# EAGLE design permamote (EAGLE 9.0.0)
AUTHOR: NEAL JACKSON; REV: B; TITLE: PERMAMOTE

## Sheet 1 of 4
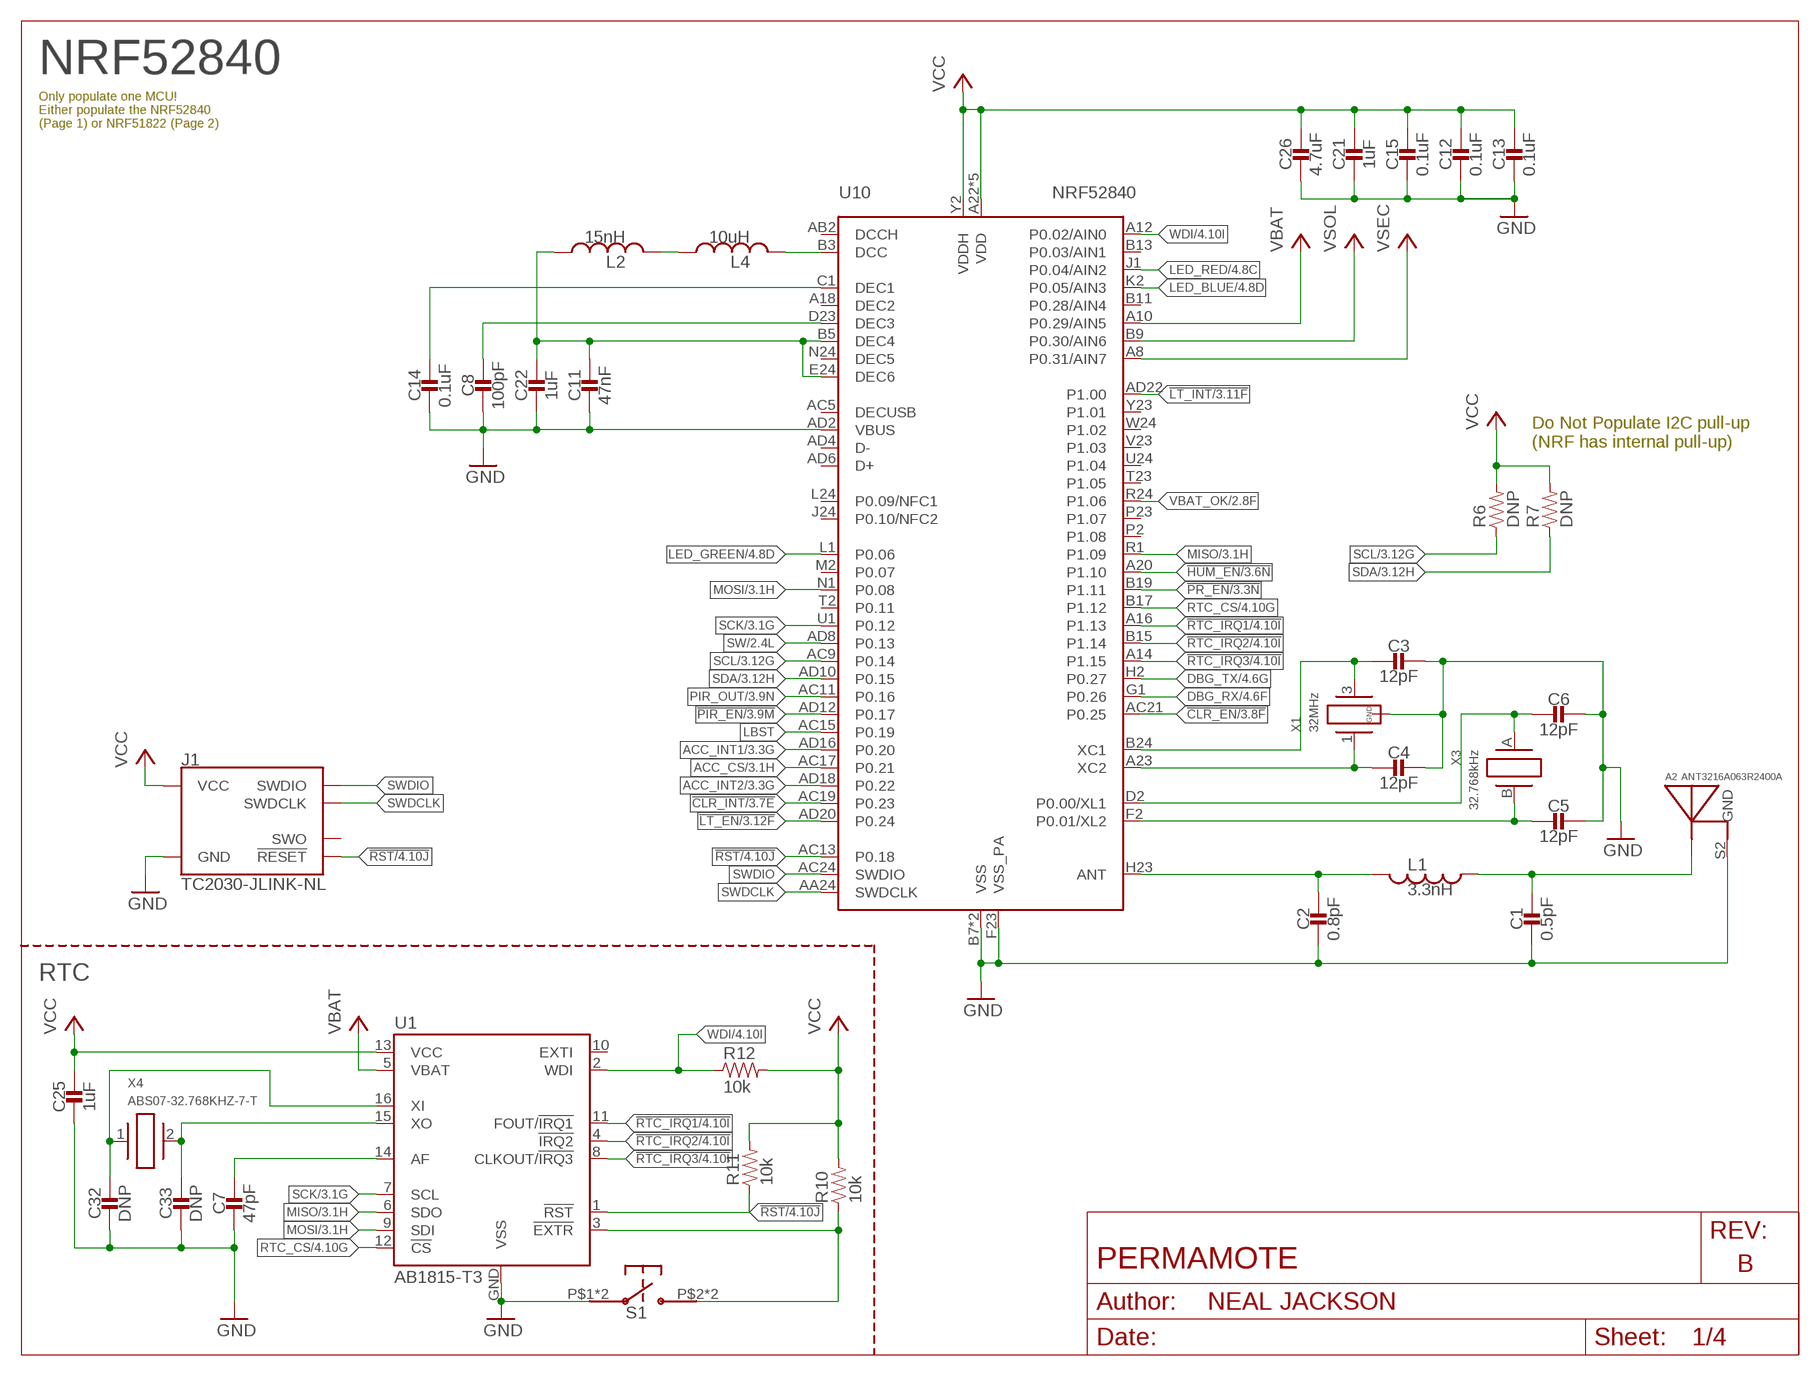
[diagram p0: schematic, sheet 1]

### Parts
A2  ANT3216A063R2400A  [ANT3216A063R2400A]
C1  0.5pF  CAPACITOR0402_CAP  [0402_CAP]
C2  0.8pF  CAPACITOR0402_CAP  [0402_CAP]
C3  12pF  CAPACITOR0402_CAP  [0402_CAP]
C4  12pF  CAPACITOR0402_CAP  [0402_CAP]
C5  12pF  CAPACITOR0402_CAP  [0402_CAP]
C6  12pF  CAPACITOR0402_CAP  [0402_CAP]
C7  47pF  CAPACITOR0402_CAP  [0402_CAP]
C8  100pF  CAPACITOR0402_CAP  [0402_CAP]
C11  47nF  CAPACITOR0402_CAP  [0402_CAP]
C12  0.1uF  CAPACITOR0402_CAP  [0402_CAP]
C13  0.1uF  CAPACITOR0402_CAP  [0402_CAP]
C14  0.1uF  CAPACITOR0402_CAP  [0402_CAP]
C15  0.1uF  CAPACITOR0402_CAP  [0402_CAP]
C21  1uF  CAPACITOR0402_CAP  [0402_CAP]
C22  1uF  CAPACITOR0402_CAP  [0402_CAP]
C25  1uF  CAPACITOR0402_CAP  [0402_CAP]
C26  4.7uF  CAPACITOR0402_CAP  [0402_CAP]
C32  DNP  CAPACITOR0402_CAP  [0402_CAP]
C33  DNP  CAPACITOR0402_CAP  [0402_CAP]
J1  TC2030-JLINK-NL  [TC2030-IDC-NL]
L1  3.3nH  INDUCTOR0402  [0402_CAP]
L2  15nH  INDUCTOR0402  [0402_CAP]
L4  10uH  INDUCTOR0603  [0603_CAP]
R6  DNP  RESISTOR0402_RES  [0402_RES]
R7  DNP  RESISTOR0402_RES  [0402_RES]
R10  10k  RESISTOR0402_RES  [0402_RES]
R11  10k  RESISTOR0402_RES  [0402_RES]
R12  10k  RESISTOR0402_RES  [0402_RES]
S1  EVQP2  [EVQP2]
U1  AB1815-T3  [QFN-16-3MM]
U10  NRF52840  [AQFN73]
X1  32MHz  7V-32.000MAHV-T  [TXC-7V]
X3  32.768kHz  ABS05-32.768KHZ-9-T  [ABS05]
X4  ABS07-32.768KHZ-7-T  [2-SMD]

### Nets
!CLR_EN: U10.AC21(P0.25) ; also sheet 3,4
!CLR_INT: U10.AC19(P0.23) ; also sheet 3,4
!HUM_EN: U10.A20(P1.10) ; also sheet 3,4
!LT_EN: U10.AD20(P0.24) ; also sheet 3,4
!LT_INT: U10.AD22(P1.00) ; also sheet 3,4
!PIR_EN: U10.AD12(P0.17) ; also sheet 3,4
!PR_EN: U10.B19(P1.11) ; also sheet 3,4
!RST: J1.3(!RESET) R11.1 U1.1(!RST) U10.AC13(P0.18) ; also sheet 4
!RTC_EXTR: R10.1 S1.P$2 S1.P$4 U1.3(!EXTR)
!RTC_IRQ1: U1.11(FOUT/!IRQ1) U10.A16(P1.13) ; also sheet 4
!RTC_IRQ2: U1.4(!IRQ2) U10.B15(P1.14) ; also sheet 4
!RTC_IRQ3: U1.8(CLKOUT/!IRQ3) U10.A14(P1.15) ; also sheet 4
ACC_CS: U10.AC17(P0.21) ; also sheet 3,4
ACC_INT1: U10.AD16(P0.20) ; also sheet 3,4
ACC_INT2: U10.AD18(P0.22) ; also sheet 3,4
DBG_RX: U10.G1(P0.26) ; also sheet 4
DBG_TX: U10.H2(P0.27) ; also sheet 4
GND: A2.S2(GND) C1.2 C2.2 C3.1 C4.1 C5.1 C6.1 C7.2 C8.2 C11.2 C12.2 C13.2 C14.2 C15.2 C21.2 C22.2 C25.2 C26.2 C32.2 C33.2 J1.5(GND) S1.P$1 S1.P$3 U1.GND(VSS) U10.AD2(VBUS) U10.B7(VSS) U10.F23(VSS_PA) U10.GND(VSS) X1.2(GND) X1.4(GND) ; also sheet 2,3,4
LBST: U10.AC15(P0.19) ; also sheet 2
LED_BLUE: U10.K2(P0.05/AIN3) ; also sheet 4
LED_GREEN: U10.L1(P0.06) ; also sheet 4
LED_RED: U10.J1(P0.04/AIN2) ; also sheet 4
MISO: U1.6(SDO) U10.R1(P1.09) ; also sheet 3,4
MOSI: U1.9(SDI) U10.N1(P0.08) ; also sheet 3,4
N$2: C14.1 U10.C1(DEC1)
N$3: C11.1 C22.1 L2.1 U10.B5(DEC4) U10.E24(DEC6)
N$4: C8.1 U10.D23(DEC3)
N$5: C2.1 L1.2 U10.H23(ANT)
N$6: A2.S1(ANTENNA) C1.1 L1.1
N$8: C3.2 U10.B24(XC1) X1.3
N$9: C4.2 U10.A23(XC2) X1.1
N$25: C7.1 U1.14(AF)
N$26: C32.1 U1.16(XI) X4.1
N$27: C33.1 U1.15(XO) X4.2
N$44: L4.2 U10.B3(DCC)
N$49: L2.2 L4.1
PIR_OUT: U10.AC11(P0.16) ; also sheet 3,4
RTC_CS: U1.12(!CS) U10.B17(P1.12) ; also sheet 4
SCK: U1.7(SCL) U10.U1(P0.12) ; also sheet 3,4
SCL: R6.1 U10.AC9(P0.14) ; also sheet 3,4
SDA: R7.1 U10.AD10(P0.15) ; also sheet 3,4
SW: U10.AD8(P0.13) ; also sheet 2,4
SWDCLK: J1.4(SWDCLK) U10.AA24(SWDCLK)
SWDIO: J1.2(SWDIO) U10.AC24(SWDIO)
VBAT: U1.5(VBAT) U10.A10(P0.29/AIN5) ; also sheet 2
VBAT_OK: U10.R24(P1.06) ; also sheet 2
VCC: C12.1 C13.1 C15.1 C21.1 C25.1 C26.1 J1.1(VCC) R6.2 R7.2 R10.2 R11.2 R12.2 U1.13(VCC) U10.A22(VDD) U10.AD14(VDD) U10.AD23(VDD) U10.B1(VDD) U10.W1(VDD) U10.Y2(VDDH) ; also sheet 2,3,4
VSEC: U10.A8(P0.31/AIN7) ; also sheet 2,4
VSOL: U10.B9(P0.30/AIN6) ; also sheet 2,4
WDI: R12.1 U1.2(WDI) U10.A12(P0.02/AIN0) ; also sheet 4
XL1: C6.2 U10.D2(P0.00/XL1) X3.A
XL2: C5.2 U10.F2(P0.01/XL2) X3.B
Unconnected: J1.6(SWO) U1.10(EXTI) U10.A18(DEC2) U10.AB2(DCCH) U10.AC5(DECUSB) U10.AD4(D-) U10.AD6(D+) U10.B11(P0.28/AIN4) U10.B13(P0.03/AIN1) U10.J24(P0.10/NFC2) U10.L24(P0.09/NFC1) U10.M2(P0.07) U10.N24(DEC5) U10.P2(P1.08) U10.P23(P1.07) U10.T2(P0.11) U10.T23(P1.05) U10.U24(P1.04) U10.V23(P1.03) U10.W24(P1.02) U10.Y23(P1.01)

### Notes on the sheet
- NRF52840
- Only populate one MCU!
  Either populate the NRF52840
  (Page 1) or NRF51822 (Page 2)
- Do Not Populate I2C pull-up
  (NRF has internal pull-up)
- RTC

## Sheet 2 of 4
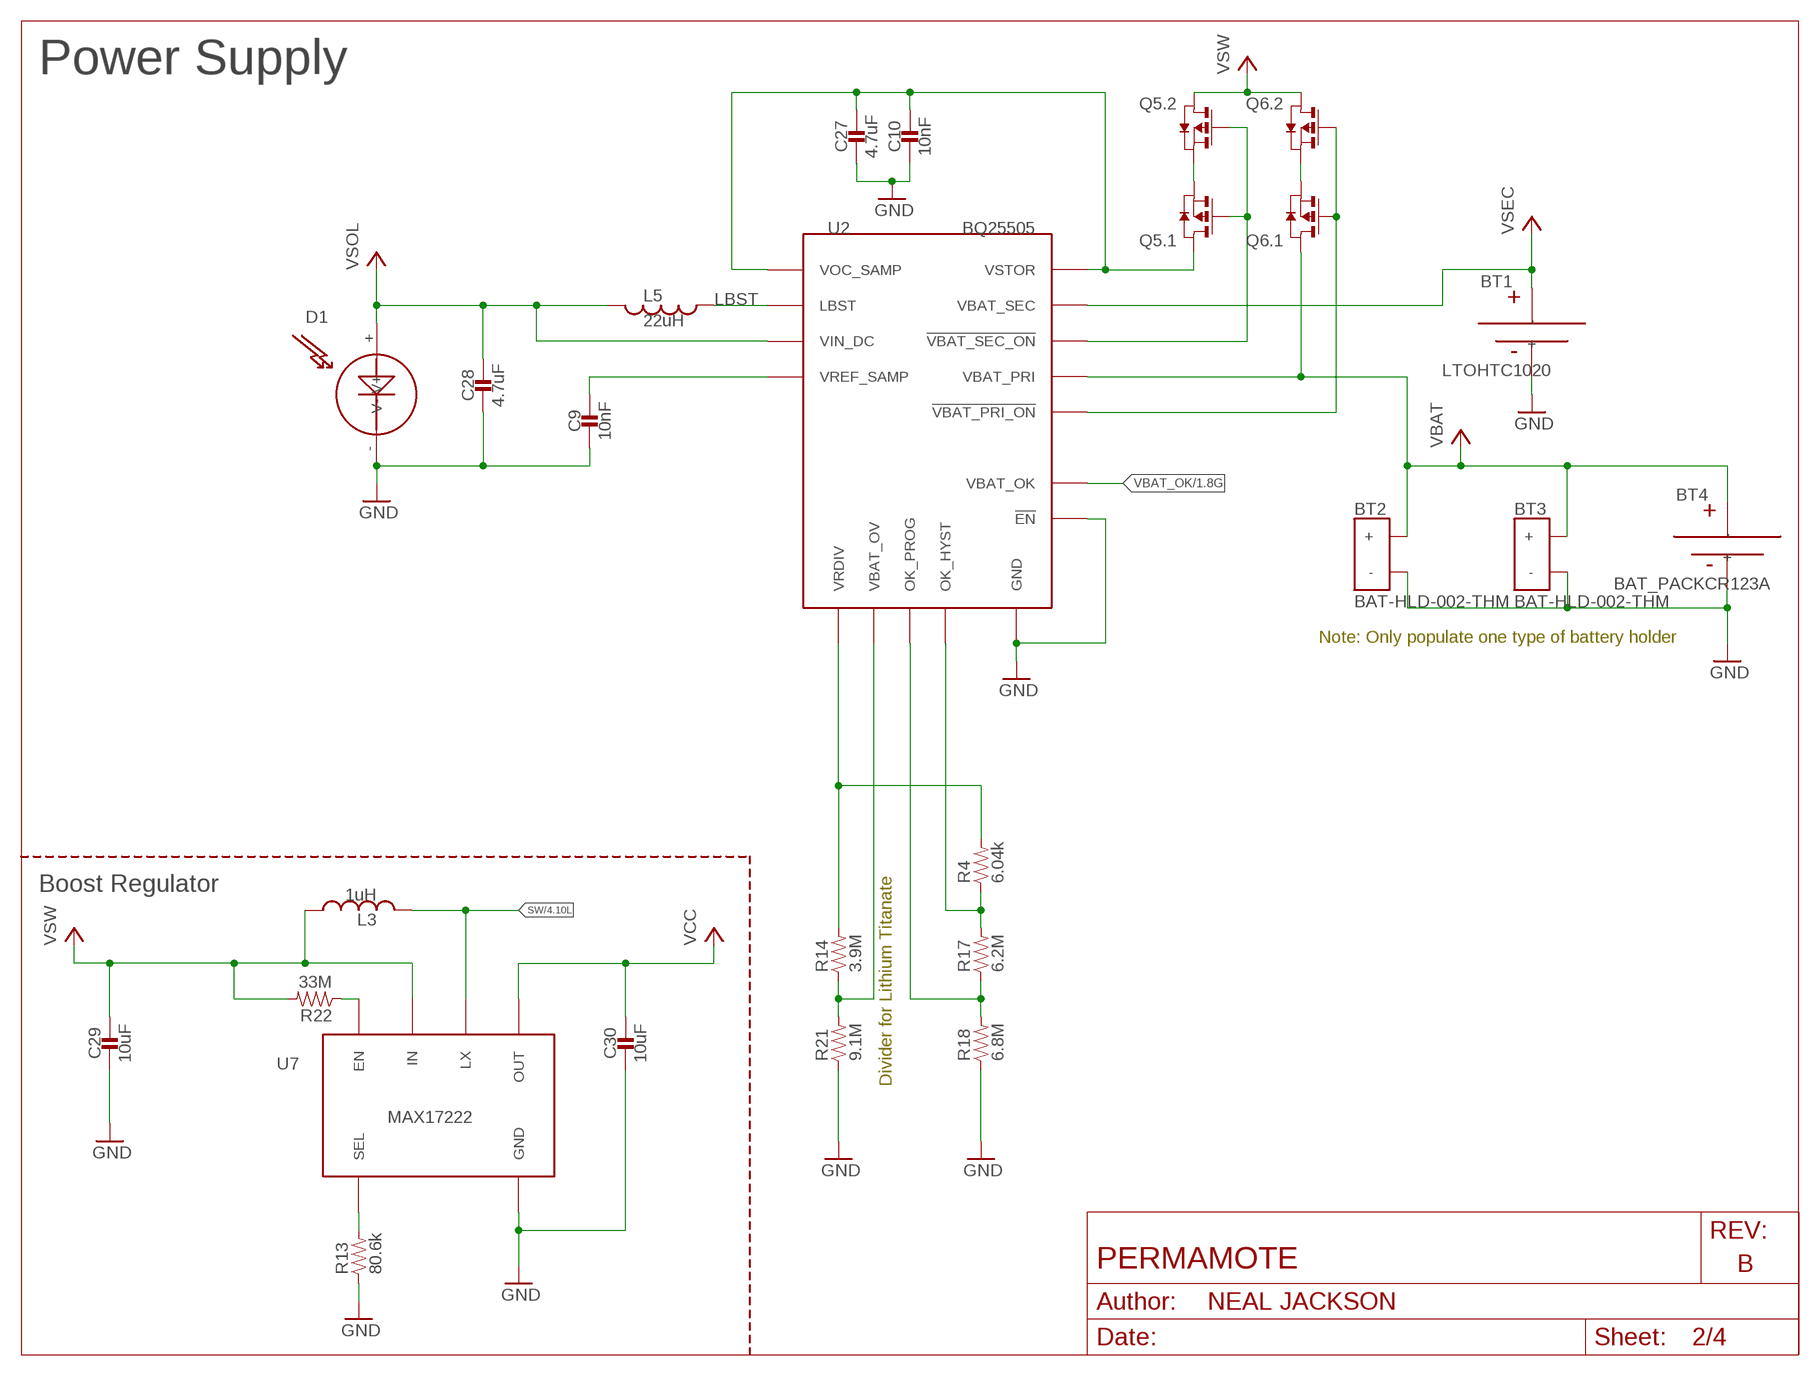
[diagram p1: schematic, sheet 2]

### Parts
BT1  LTOHTC1020  [1020]
BT2  BAT-HLD-002-THM  [BAT-HLD-002-THM]
BT3  BAT-HLD-002-THM  [BAT-HLD-002-THM]
BT4  BAT_PACKCR123A  [BH123A]
C9  10nF  CAPACITOR0402_CAP  [0402_CAP]
C10  10nF  CAPACITOR0402_CAP  [0402_CAP]
C27  4.7uF  CAPACITOR0402_CAP  [0402_CAP]
C28  4.7uF  CAPACITOR0402_CAP  [0402_CAP]
C29  10uF  CAPACITOR0603_CAP  [0603_CAP]
C30  10uF  CAPACITOR0603_CAP  [0603_CAP]
D1  SOLARCELLHOLES  [SOLAR_HOLES]
L3  1uH  INDUCTORIHL  [IHL-1212BZ-11]
L5  22uH  INDUCTOR74437324220  [74437324220]
Q5  PMDXB950UPEL  [XDFN-6]
Q6  PMDXB950UPEL  [XDFN-6]
R4  6.04k  RESISTOR0402_RES  [0402_RES]
R13  80.6k  RESISTOR0603_RES  [0603-RES]
R14  3.9M  RESISTOR0402_RES  [0402_RES]
R17  6.2M  RESISTOR0402_RES  [0402_RES]
R18  6.8M  RESISTOR0402_RES  [0402_RES]
R21  9.1M  RESISTOR0402_RES  [0402_RES]
R22  33M  RESISTOR0603_RES  [0603-RES]
U2  BQ25505  [S-PVQFN-N20-RGR]
U7  MAX17222  [UDFN-6-MAXIM]

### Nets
!VBAT_PRI_ON: Q6.2(.1:G) Q6.5(.2:G) U2.10(!VBAT_PRI_ON)
!VBAT_SEC_ON: Q5.2(.1:G) Q5.5(.2:G) U2.9(!VBAT_SEC_ON)
GND: BT1.- BT2.GND(-) BT3.GND(-) BT4.- C9.2 C10.2 C27.2 C28.2 C29.2 C30.2 D1.-(V-) R13.1 R18.1 R21.1 U2.1(GND) U2.5(!EN) U2.6(GND) U2.15(GND) U2.16(GND) U2.17(GND) U2.PAD(GND) U7.3(GND) ; also sheet 1,3,4
LBST: L5.P$1 U2.20(LBST) ; also sheet 1
N$12: R13.2 U7.4(SEL)
N$14: R22.1 U7.6(EN)
N$18: R14.1 R21.2 U2.7(VBAT_OV)
N$32: R4.2 R14.2 U2.8(VRDIV)
N$45: Q5.1(.1:S) Q5.4(.2:S)
N$53: Q6.1(.1:S) Q6.4(.2:S)
N$57: R17.1 R18.2 U2.12(OK_PROG)
N$58: R4.1 R17.2 U2.11(OK_HYST)
SW: L3.P$2 U7.2(LX) ; also sheet 1,4
VBAT: BT2.POS1(+) BT2.POS2(+) BT2.POS3(+) BT2.POS4(+) BT3.POS1(+) BT3.POS2(+) BT3.POS3(+) BT3.POS4(+) BT4.+ Q6.6(.1:D) U2.14(VBAT_PRI) ; also sheet 1
VBAT_OK: U2.13(VBAT_OK) ; also sheet 1
VCC: C30.1 U7.1(OUT) ; also sheet 1,3,4
VOC_SAMP_VSTOR: C10.1 C27.1 Q5.6(.1:D) U2.3(VOC_SAMP) U2.19(VSTOR)
VREF_SAMP: C9.1 U2.4(VREF_SAMP)
VSEC: BT1.+ U2.18(VBAT_SEC) ; also sheet 1,4
VSOL: C28.1 D1.+(V+) L5.P$2 U2.2(VIN_DC) ; also sheet 1,4
VSW: C29.1 L3.P$1 Q5.3(.2:D) Q6.3(.2:D) R22.2 U7.5(IN)

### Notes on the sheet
- Power Supply
- Note: Only populate one type of battery holder
- Boost Regulator
- Divider for Lithium Titanate

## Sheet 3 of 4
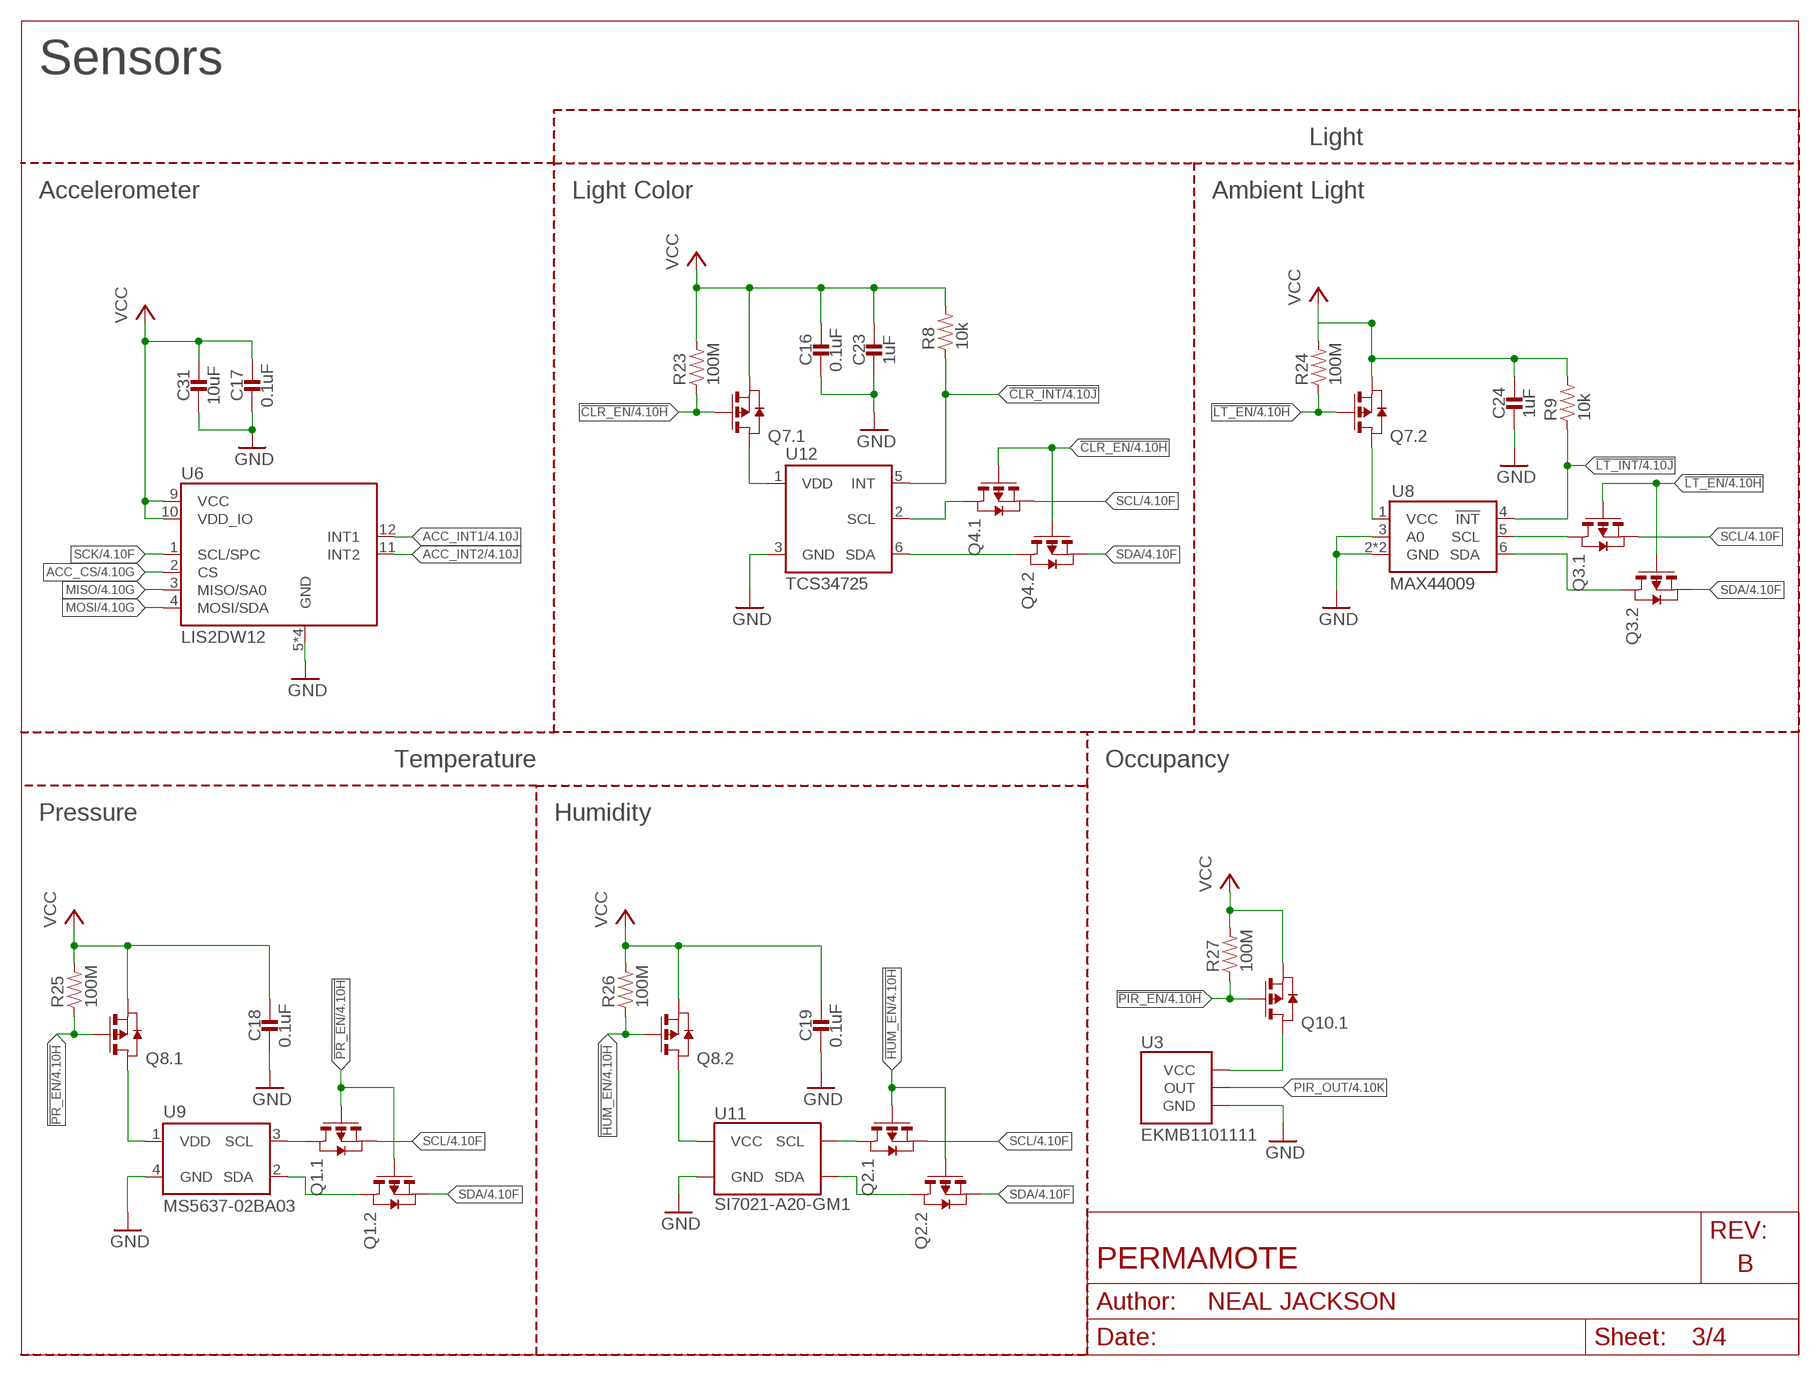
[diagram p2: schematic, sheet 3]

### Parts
C16  0.1uF  CAPACITOR0402_CAP  [0402_CAP]
C17  0.1uF  CAPACITOR0402_CAP  [0402_CAP]
C18  0.1uF  CAPACITOR0402_CAP  [0402_CAP]
C19  0.1uF  CAPACITOR0402_CAP  [0402_CAP]
C23  1uF  CAPACITOR0402_CAP  [0402_CAP]
C24  1uF  CAPACITOR0402_CAP  [0402_CAP]
C31  10uF  CAPACITOR0603_CAP  [0603_CAP]
Q1  PMDXB950UPEL  [XDFN-6]
Q2  PMDXB950UPEL  [XDFN-6]
Q3  PMDXB950UPEL  [XDFN-6]
Q4  PMDXB950UPEL  [XDFN-6]
Q7  PMDXB950UPEL  [XDFN-6]
Q8  PMDXB950UPEL  [XDFN-6]
Q10  PMDXB950UPEL  [XDFN-6]
R8  10k  RESISTOR0402_RES  [0402_RES]
R9  10k  RESISTOR0402_RES  [0402_RES]
R23  100M  RESISTOR0402_RES  [0402_RES]
R24  100M  RESISTOR0402_RES  [0402_RES]
R25  100M  RESISTOR0402_RES  [0402_RES]
R26  100M  RESISTOR0402_RES  [0402_RES]
R27  100M  RESISTOR0402_RES  [0402_RES]
U3  EKMB1101111  [AMN2]
U6  LIS2DW12  [LGA-12]
U8  MAX44009  [UDFN-6-EXPOSED]
U9  MS5637-02BA03  [4-SMD]
U11  SI7021-A20-GM1  [DFN-6/3MM]
U12  TCS34725  [FN-6]

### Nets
!CLR_EN: Q4.2(.1:G) Q4.5(.2:G) Q7.2(.1:G) R23.1 ; also sheet 1,4
!CLR_INT: R8.1 U12.5(INT) ; also sheet 1,4
!HUM_EN: Q2.2(.1:G) Q2.5(.2:G) Q8.5(.2:G) R26.1 ; also sheet 1,4
!LT_EN: Q3.2(.1:G) Q3.5(.2:G) Q7.5(.2:G) R24.1 ; also sheet 1,4
!LT_INT: R9.1 U8.4(!INT) ; also sheet 1,4
!PIR_EN: Q10.2(.1:G) R27.1 ; also sheet 1,4
!PR_EN: Q1.2(.1:G) Q1.5(.2:G) Q8.2(.1:G) R25.1 ; also sheet 1,4
ACC_CS: U6.2(CS) ; also sheet 1,4
ACC_INT1: U6.12(INT1) ; also sheet 1,4
ACC_INT2: U6.11(INT2) ; also sheet 1,4
GND: C16.2 C17.2 C18.2 C19.2 C23.2 C24.2 C31.2 U3.GND U6.5(GND) U6.6(GND) U6.7(GND) U6.8(GND) U8.2(GND) U8.3(A0) U8.EP(GND) U9.4(GND) U11.2(GND) U12.3(GND) ; also sheet 1,2,4
MISO: U6.3(MISO/SA0) ; also sheet 1,4
MOSI: U6.4(MOSI/SDA) ; also sheet 1,4
N$20: Q7.3(.2:D) U8.1(VCC)
N$21: Q8.6(.1:D) U9.1(VDD)
N$22: Q8.3(.2:D) U11.5(VCC)
N$23: Q10.6(.1:D) U3.VCC
N$31: Q7.6(.1:D) U12.1(VDD)
N$34: Q1.6(.1:D) U9.3(SCL)
N$41: Q1.3(.2:D) U9.2(SDA)
N$48: Q2.3(.2:D) U11.1(SDA)
N$50: Q2.6(.1:D) U11.6(SCL)
N$51: Q3.3(.2:D) U8.6(SDA)
N$52: Q3.6(.1:D) U8.5(SCL)
N$54: Q4.3(.2:D) U12.6(SDA)
N$55: Q4.6(.1:D) U12.2(SCL)
PIR_OUT: U3.OUT ; also sheet 1,4
SCK: U6.1(SCL/SPC) ; also sheet 1,4
SCL: Q1.1(.1:S) Q2.1(.1:S) Q3.1(.1:S) Q4.1(.1:S) ; also sheet 1,4
SDA: Q1.4(.2:S) Q2.4(.2:S) Q3.4(.2:S) Q4.4(.2:S) ; also sheet 1,4
VCC: C16.1 C17.1 C18.1 C19.1 C23.1 C24.1 C31.1 Q7.1(.1:S) Q7.4(.2:S) Q8.1(.1:S) Q8.4(.2:S) Q10.1(.1:S) R8.2 R9.2 R23.2 R24.2 R25.2 R26.2 R27.2 U6.9(VCC) U6.10(VDD_IO) ; also sheet 1,2,4
Unconnected: Q10.3(.2:D) Q10.4(.2:S) Q10.5(.2:G)

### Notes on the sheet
- Sensors
- Light
- Accelerometer | Light Color | Ambient Light
- Temperature | Occupancy
- Pressure | Humidity

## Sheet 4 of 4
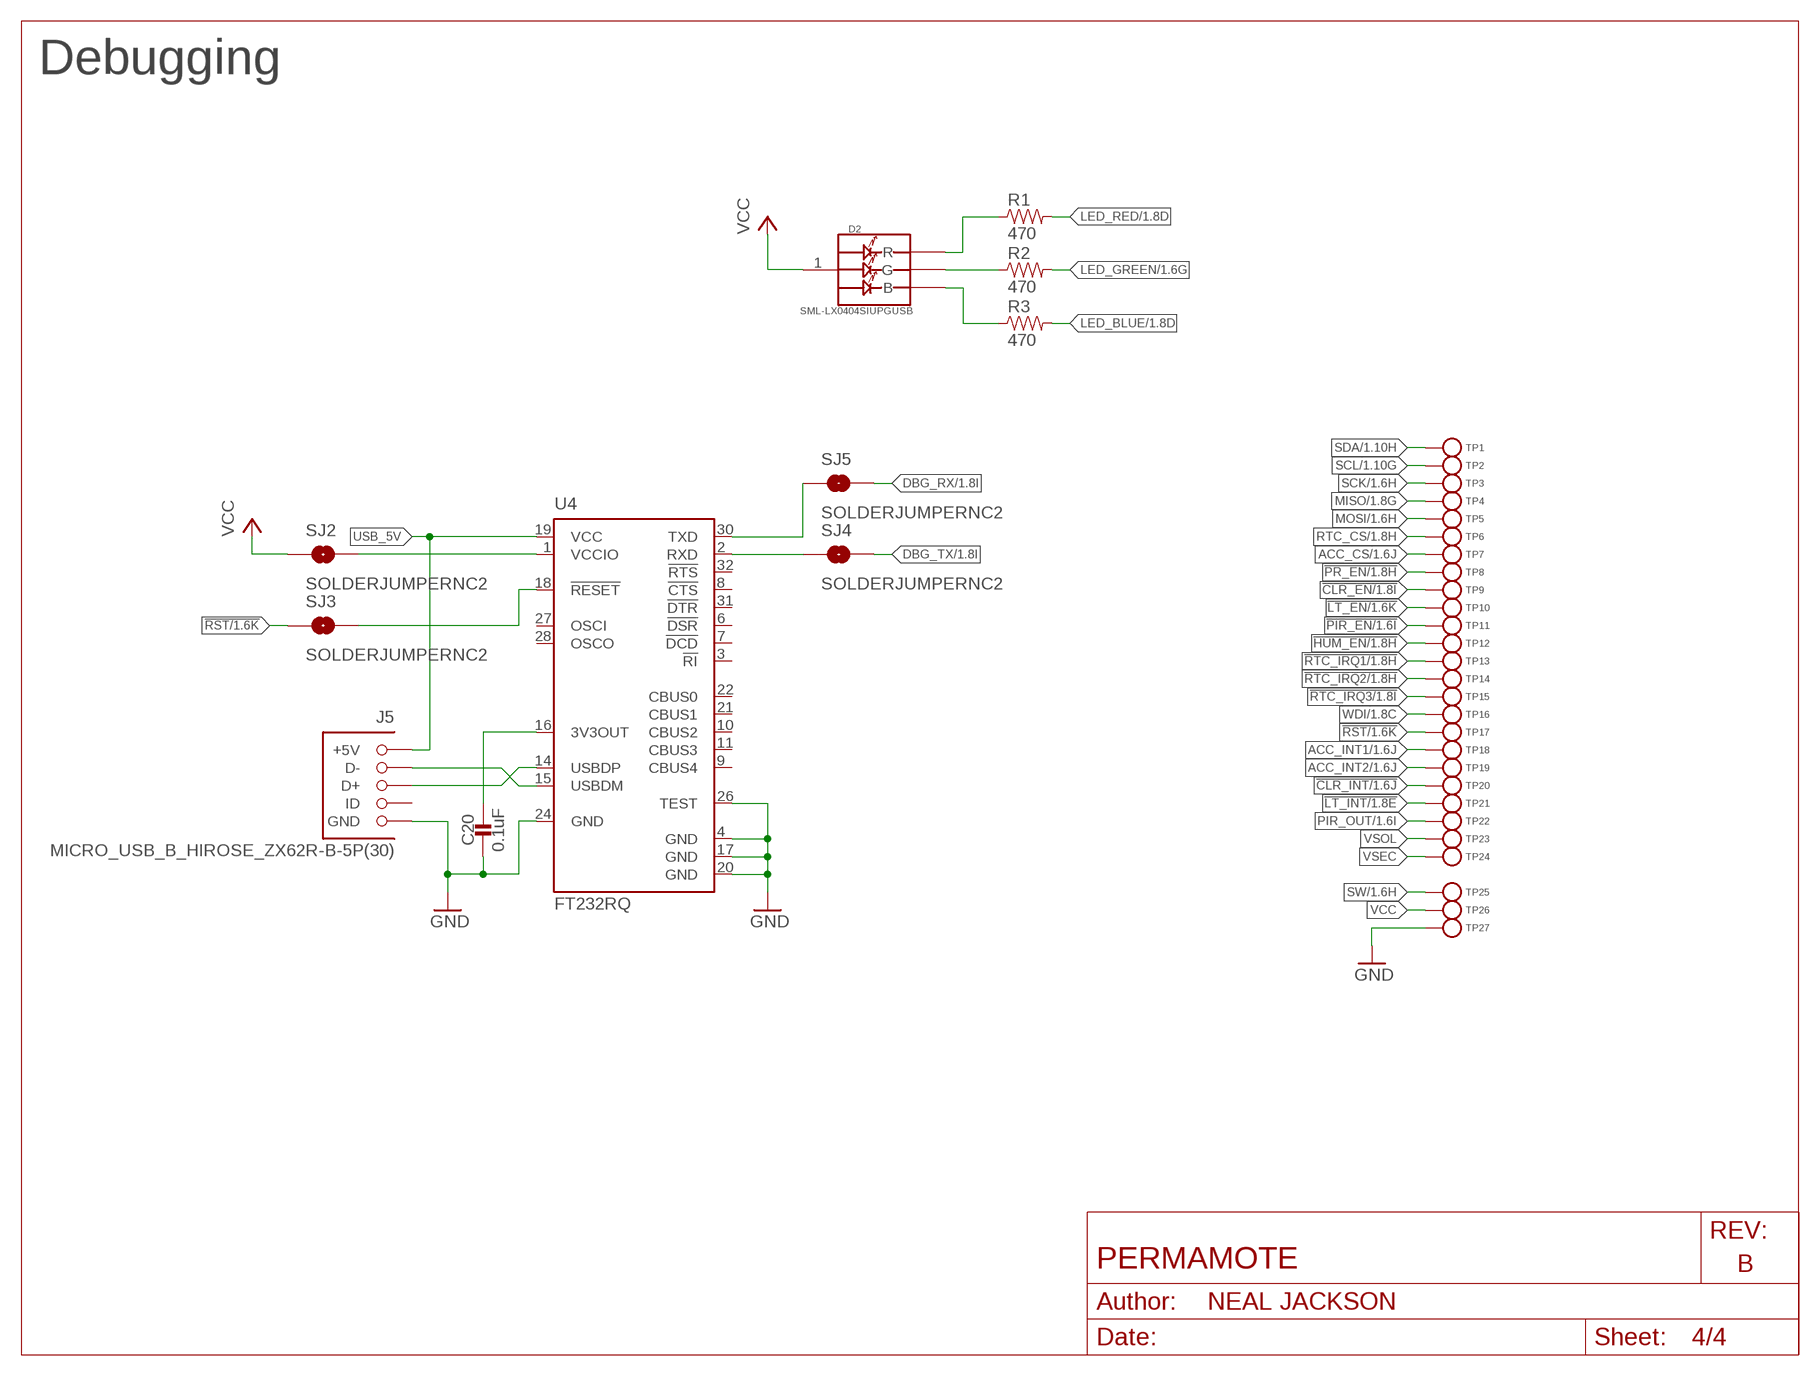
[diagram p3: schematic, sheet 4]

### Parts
C20  0.1uF  CAPACITOR0402_CAP  [0402_CAP]
D2  SML-LX0404SIUPGUSB  [1MM_SQ_4PAD]
J5  MICRO_USB_B_HIROSE_ZX62R-B-5P(30)  [MICRO_USB_B_HIROSE_ZX62R-B-5P(30)]
R1  470  RESISTOR0402_RES  [0402_RES]
R2  470  RESISTOR0402_RES  [0402_RES]
R3  470  RESISTOR0402_RES  [0402_RES]
SJ2  SOLDERJUMPERNC2  [SJ_2S-NOTRACE]
SJ3  SOLDERJUMPERNC2  [SJ_2S-NOTRACE]
SJ4  SOLDERJUMPERNC2  [SJ_2S-NOTRACE]
SJ5  SOLDERJUMPERNC2  [SJ_2S-NOTRACE]
TP1  TEST-POINT  [PAD.03X.03]
TP2  TEST-POINT  [PAD.03X.03]
TP3  TEST-POINT  [PAD.03X.03]
TP4  TEST-POINT  [PAD.03X.03]
TP5  TEST-POINT  [PAD.03X.03]
TP6  TEST-POINT  [PAD.03X.03]
TP7  TEST-POINT  [PAD.03X.03]
TP8  TEST-POINT  [PAD.03X.03]
TP9  TEST-POINT  [PAD.03X.03]
TP10  TEST-POINT  [PAD.03X.03]
TP11  TEST-POINT  [PAD.03X.03]
TP12  TEST-POINT  [PAD.03X.03]
TP13  TEST-POINT  [PAD.03X.03]
TP14  TEST-POINT  [PAD.03X.03]
TP15  TEST-POINT  [PAD.03X.03]
TP16  TEST-POINT  [PAD.03X.03]
TP17  TEST-POINT  [PAD.03X.03]
TP18  TEST-POINT  [PAD.03X.03]
TP19  TEST-POINT  [PAD.03X.03]
TP20  TEST-POINT  [PAD.03X.03]
TP21  TEST-POINT  [PAD.03X.03]
TP22  TEST-POINT  [PAD.03X.03]
TP23  TEST-POINT  [PAD.03X.03]
TP24  TEST-POINT  [PAD.03X.03]
TP25  TEST-POINT  [PAD.03X.03]
TP26  TEST-POINT  [PAD.03X.03]
TP27  TEST-POINT  [PAD.03X.03]
U4  FT232RQ  [QFN32]

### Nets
!CLR_EN: TP9.P$1(TESTPOINT) ; also sheet 1,3
!CLR_INT: TP20.P$1(TESTPOINT) ; also sheet 1,3
!FTDI_RESET: SJ3.2 U4.18(!RESET)
!HUM_EN: TP12.P$1(TESTPOINT) ; also sheet 1,3
!LT_EN: TP10.P$1(TESTPOINT) ; also sheet 1,3
!LT_INT: TP21.P$1(TESTPOINT) ; also sheet 1,3
!PIR_EN: TP11.P$1(TESTPOINT) ; also sheet 1,3
!PR_EN: TP8.P$1(TESTPOINT) ; also sheet 1,3
!RST: SJ3.1 TP17.P$1(TESTPOINT) ; also sheet 1
!RTC_IRQ1: TP13.P$1(TESTPOINT) ; also sheet 1
!RTC_IRQ2: TP14.P$1(TESTPOINT) ; also sheet 1
!RTC_IRQ3: TP15.P$1(TESTPOINT) ; also sheet 1
ACC_CS: TP7.P$1(TESTPOINT) ; also sheet 1,3
ACC_INT1: TP18.P$1(TESTPOINT) ; also sheet 1,3
ACC_INT2: TP19.P$1(TESTPOINT) ; also sheet 1,3
D+: J5.3(D+) U4.14(USBDP)
D-: J5.2(D-) U4.15(USBDM)
DBG_RX: SJ5.2 ; also sheet 1
DBG_TX: SJ4.2 ; also sheet 1
FTDI_VCCIO: SJ2.2 U4.1(VCCIO)
GND: C20.2 J5.5(GND) TP27.P$1(TESTPOINT) U4.4(GND) U4.17(GND) U4.20(GND) U4.24(GND) U4.26(TEST) ; also sheet 1,2,3
LED_BLUE: R3.2 ; also sheet 1
LED_GREEN: R2.2 ; also sheet 1
LED_RED: R1.2 ; also sheet 1
MISO: TP4.P$1(TESTPOINT) ; also sheet 1,3
MOSI: TP5.P$1(TESTPOINT) ; also sheet 1,3
N$13: C20.1 U4.16(3V3OUT)
N$15: D2.2(R) R1.1
N$17: D2.4(G) R2.1
N$19: D2.3(B) R3.1
PIR_OUT: TP22.P$1(TESTPOINT) ; also sheet 1,3
RTC_CS: TP6.P$1(TESTPOINT) ; also sheet 1
RXD: SJ4.1 U4.2(RXD)
SCK: TP3.P$1(TESTPOINT) ; also sheet 1,3
SCL: TP2.P$1(TESTPOINT) ; also sheet 1,3
SDA: TP1.P$1(TESTPOINT) ; also sheet 1,3
SW: TP25.P$1(TESTPOINT) ; also sheet 1,2
TXD: SJ5.1 U4.30(TXD)
USB_5V: J5.1(+5V) U4.19(VCC)
VCC: D2.1(VDD) SJ2.1 TP26.P$1(TESTPOINT) ; also sheet 1,2,3
VSEC: TP24.P$1(TESTPOINT) ; also sheet 1,2
VSOL: TP23.P$1(TESTPOINT) ; also sheet 1,2
WDI: TP16.P$1(TESTPOINT) ; also sheet 1
Unconnected: J5.4(ID) U4.3(!RI) U4.6(!DSR) U4.7(!DCD) U4.8(!CTS) U4.9(CBUS4) U4.10(CBUS2) U4.11(CBUS3) U4.21(CBUS1) U4.22(CBUS0) U4.27(OSCI) U4.28(OSCO) U4.31(!DTR) U4.32(!RTS)

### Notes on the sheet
- Debugging

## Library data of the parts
A2 = chips:ANT3216A063R2400A: Yageo 2.4GHz; DIGIKEY: 311-1542-1-ND; MANUFACTURER: YAGEO; MPN: ANT3216A063R2400A
BT1 = batteries:LTOHTC
BT2 BT3 = batteries:BAT-HLD-002-THM: RETAINER BATT CR2016 PC PINS; DIGIKEY: BAT-HLD-001-THM-ND; MOUSER: 712-BAT-HLD-001-THM; MPN: BAT-HLD-001-THM
BT4 = batteries:BAT_PACK: collection of battery footprints; DIGIKEY: BH123A-ND; MANUFACTURER: MPD; MPN: BH123A
C1 = passives:CAPACITOR: SMD Capacitor; DIGIKEY: 490-6264-1-ND; MPN: GRM1555C1HR50WA01D
C2 = passives:CAPACITOR: SMD Capacitor; DIGIKEY: 490-6269-1-ND; MPN: GRM1555C1HR80BA01D
C3-C6 = passives:CAPACITOR: SMD Capacitor; DIGIKEY: 490-6197-1-ND; MPN: GRM1555C1H120GA01D
C7 = passives:CAPACITOR: SMD Capacitor; DIGIKEY: 490-5942-1-ND; MPN: GRM1555C1H470JA01D
C8 = passives:CAPACITOR: SMD Capacitor; DIGIKEY: 490-5922-1-ND; MPN: GRM1555C1H101JA01D
C9 C10 = passives:CAPACITOR: SMD Capacitor; DIGIKEY: 490-4516-1-ND; MPN: GRM155R71H103KA88D
C11 = passives:CAPACITOR: SMD Capacitor; DIGIKEY: 445-1264-1-ND; MPN: C1005X7R1C473K050BC
C12-C20 = passives:CAPACITOR: SMD Capacitor; DIGIKEY: 490-6328-1-ND; MPN: GRM155R71C104KA88J
C21-C25 = passives:CAPACITOR: SMD Capacitor; DIGIKEY: 490-7195-1-ND; MPN: GRM155R70G105KA12D
C26-C28 = passives:CAPACITOR: SMD Capacitor; DIGIKEY: 445-5947-1-ND; MPN: C1005X5R0J475K050BC
C29-C31 = passives:CAPACITOR: SMD Capacitor; DIGIKEY: 490-3896-1-ND; MPN: GRM188R60J106ME47D
C32 C33 = passives:CAPACITOR: SMD Capacitor
D1 = permamote:SOLARCELL: Generic solar cell; DIGIKEY: 869-1001-ND; MPN: AM-1454CA
D2 = leds:SML-LX0404SIUPGUSB: 1mm^2 RGB LED; DIGIKEY: 67-2125-1-ND; MANUFACTURER: Lumex Opto; MPN: SML-LX0404SIUPGUSB
J1 = connector:TC2030-JLINK
J5 = connector:MICRO_USB_B_HIROSE_ZX62R-B-5P(30): USB Micro B Connector Rounded side is up.; DIGIKEY: H125274CT-ND; MOUSER: 798-ZX62R-B-5P30; MPN: ZX62R-B-5P(30); NEWARK: 84Y6712
L1 = passives:INDUCTOR: A very specific inductor; DIGIKEY: 535-10426-1-ND; MPN: AISC-0402-3N3J-T
L2 = passives:INDUCTOR: A very specific inductor; DIGIKEY: 587-1521-1-ND; MPN: HK100515NJ-T
L3 = passives:INDUCTOR: A very specific inductor; DIGIKEY: 541-1319-1-ND; MANUFACTURER: Vishay Dale; MPN: IHLP1212BZER1R0M11
L4 = passives:INDUCTOR: A very specific inductor; DIGIKEY: 490-4025-1-ND; MPN: LQM18FN100M00D
L5 = passives:INDUCTOR: A very specific inductor; DIGIKEY: 732-3340-1-ND; MPN: 74437324220
Q1-Q8 Q10 = fets:PMDXB950UPEL: 20 V 500mA, dual P-channel Trench MOSFET; DIGIKEY: 1727-2601-1-ND; MANUFACTURER: NEXPERIA; MPN: PMDXB950UPELZ
R1-R3 = passives:RESISTOR: Resistor; DIGIKEY: 311-470JRCT-ND; MPN: RC0402JR-07470RL
R4 = passives:RESISTOR: Resistor; DIGIKEY: YAG2293CT-ND; MPN: RC0402FR-076K04L
R6-R12 = passives:RESISTOR: Resistor; DIGIKEY: 311-10KJRCT-ND; MPN: RC0402JR-0710KL
R13 = passives:RESISTOR: Resistor; DIGIKEY: 311-80.6KHRCT-ND; MPN: RC0603FR-0780K6L
R14 = passives:RESISTOR: Resistor; DIGIKEY: YAG3301CT-ND; MPN: RC0402JR-073M9L
R17 = passives:RESISTOR: Resistor; DIGIKEY: YAG3309CT-ND; MPN: RC0402JR-076M2L
R18 = passives:RESISTOR: Resistor; DIGIKEY: YAG3310CT-ND; MPN: RC0402JR-076M8L
R21 = passives:RESISTOR: Resistor; DIGIKEY: YAG3322CT-ND; MPN: RC0402JR-079M1L
R22 = passives:RESISTOR: Resistor; DIGIKEY: HMC0603JT33M0CT-ND; MPN: HMC0603JT33M0
R23-R27 = passives:RESISTOR: Resistor; DIGIKEY: 541-100MAHCT-ND; MPN: HMC0402JT100M
S1 = switches:EVQP2: SWITCH TACTILE SPST-NO 0.02A 15V; DIGIKEY: P11084SCT-ND; MPN: EVQ-P2K02Q
SJ2-SJ5 = SparkFun-Passives:SOLDERJUMPER: Solder Jumper
TP1-TP27 = headers:TEST-POINT
U1 = chips:AB1815-T3: Ultra-low current RTC. 55nA quiescent @ 3V. 1.5-3.6V input.; DIGIKEY: 535-11936-1-ND; MANUFACTURER: Abracon; MPN: AB1815-T3
U2 = chips:BQ25505: EH front end for switching between primary and secondary cells; DIGIKEY: 296-37078-1-ND; MANUFACTURER: TI; MPN: BQ25505RGRR
U3 = chips:EKMB: Passive infrared human detection sensor with built-in amp.; DIGIKEY: 255-3065-ND; MANUFACTURER: PANASONIC; MPN: EKMB1101111
U4 = ftdichip:FT232R: Source: http://www.ftdichip.com/Documents/DataSheets/DS_FT232R_v104.pdf; MPN: FT232RQ; OC_FARNELL: 1146033; OC_NEWARK: 91K9919
U6 = chips:LIS2DW12: ultra low power 3 axis accelerometer; MANUFACTURER: STMicroelectronics; MOUSER: 511-LIS2DW12TR; MPN: LIS2DW12TR
U7 = chips:MAX17222: Very high efficiency, very low power boost converter suitable for EH applications; DIGIKEY: MAX17222ELT+TCT-ND; MANUFACTURER: MAXIM INTEGRATED; MPN: MAX17222ELT+T
U8 = chips:MAX44009: low power ambient light sensor; DIGIKEY: MAX44009EDT+TCT-ND; MANUFACTURER: MAXIM; MPN: MAX44009EDT+T
U9 = chips:MS5637-02BA03: low power pressure sensor; DIGIKEY: 223-1199-1-ND; MANUFACTURER: TE CONNECTIVITY; MPN: MS563702BA03-50
U10 = chips:NRF52840: ultra-low power 2.4 GHz wireless system on chip (SoC) integrating a multiprotocol 2.4 GHz transceiver, an ARM® Cortex®-M4F CPU.; DIGIKEY: 1490-1071-1-ND; MANUFACTURER: NORIDIC SEMICONDUCTOR; MPN: NRF52840
U11 = chips:SI7021: IC TEMP SENSOR RH 2% DFN; DIGIKEY: 336-3141-ND; MOUSER: 634-SI7021-A20-GM1; MPN: SI7021-A20-GM1
U12 = chips:TCS34725: Color Light-to-Digital Converter with IR Filter; DIGIKEY: TCS34725FNCT-ND; MPN: TCS34725FN
X1 = crystals:7V: TXC CRYSTAL SMD; DIGIKEY: 887-2568-1-ND; MANUFACTURER: TXC CORPORATION; MPN: 7M-32.000MAHV-T
X3 = crystals:ABS05-32.768KHZ: 32.768kHz Crystal; DIGIKEY: 535-11897-1-ND; MANUFACTURER: Abracon; MPN: ABS05-32.768KHZ-9-T
X4 = crystals:ABS07-32.768KHZ: 32.768kHz Crystal; DIGIKEY: 535-9543-1-ND; MANUFACTURER: ABRACON; MPN: ABS07-32.768KHZ-7-T

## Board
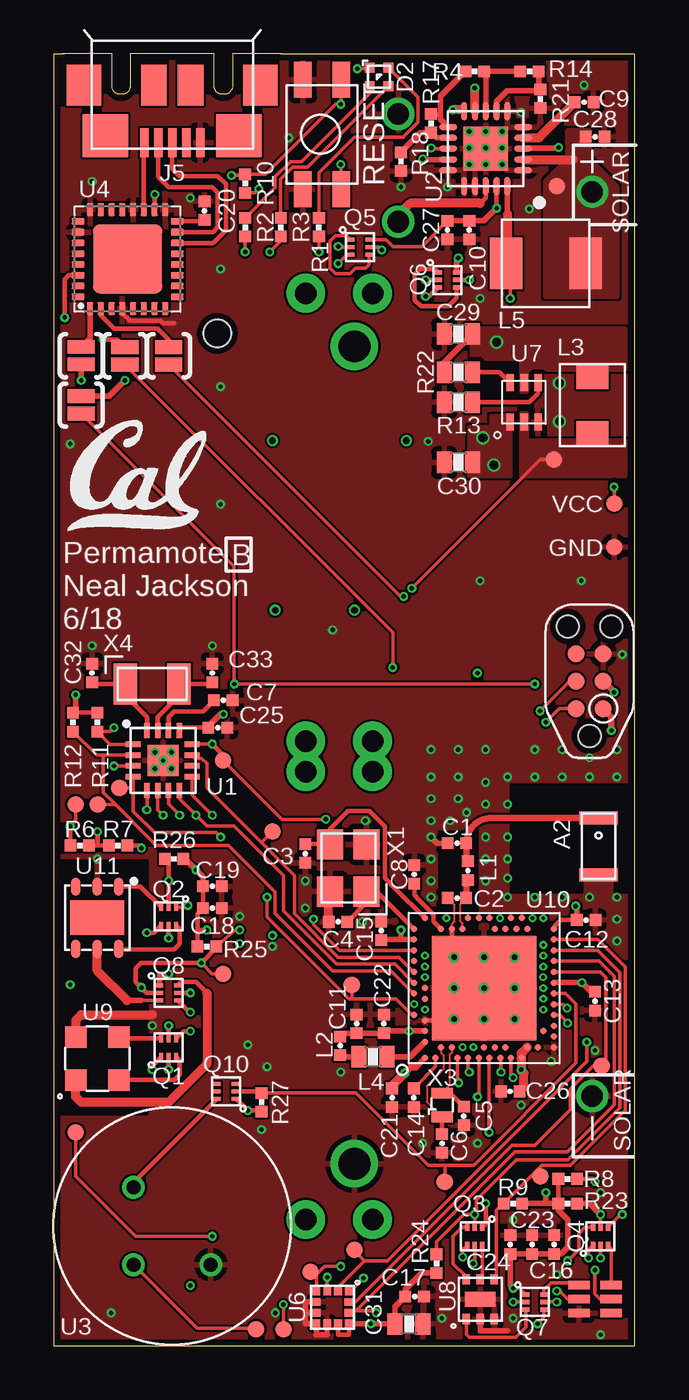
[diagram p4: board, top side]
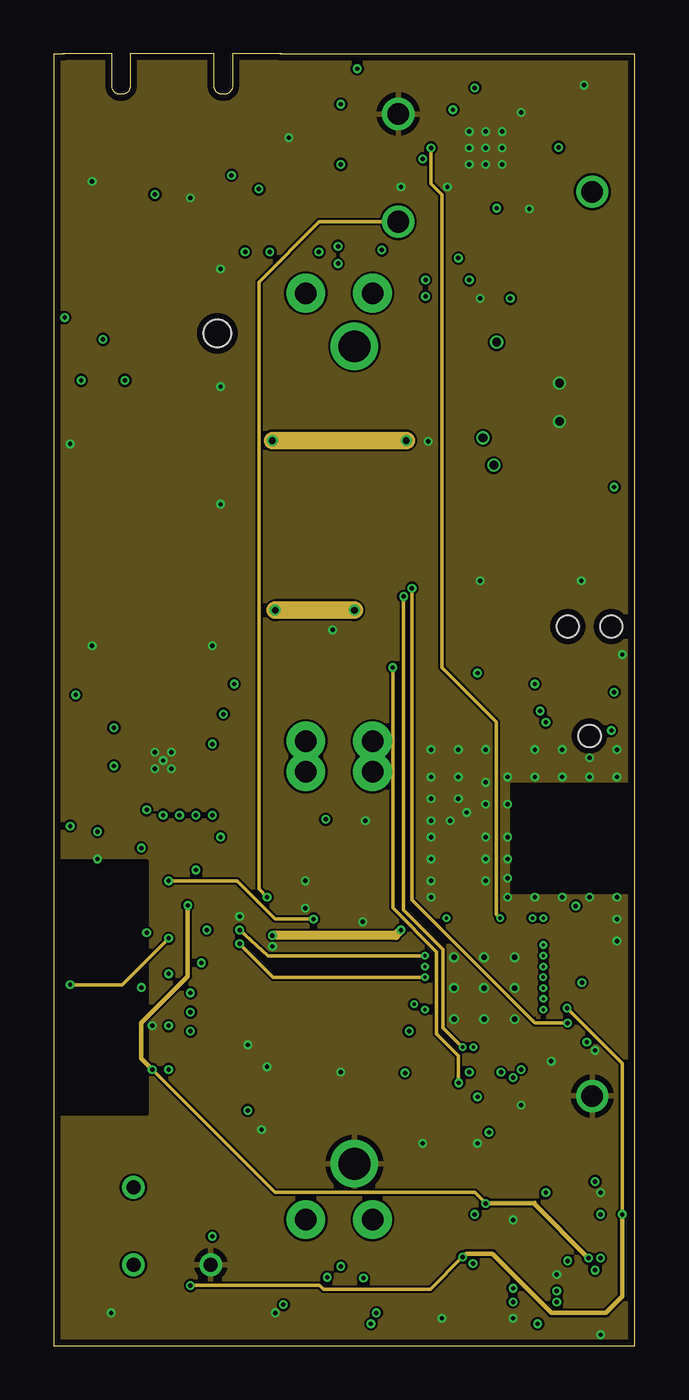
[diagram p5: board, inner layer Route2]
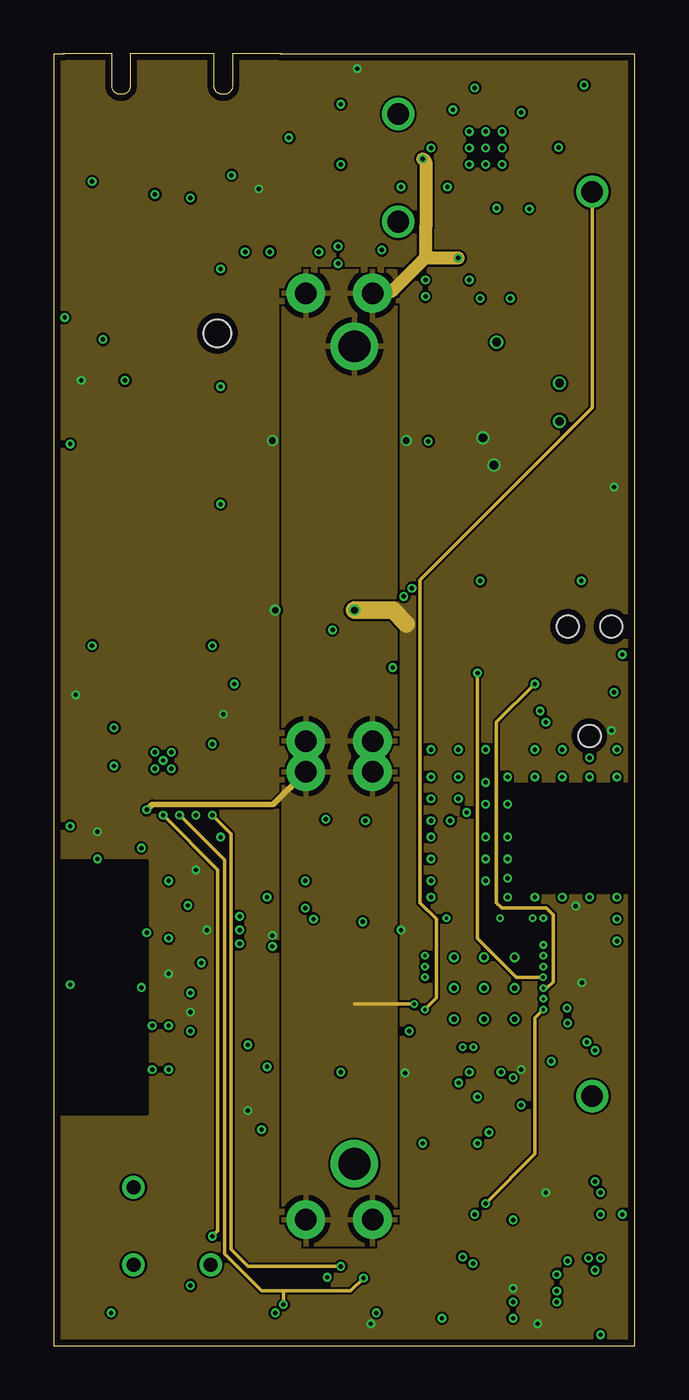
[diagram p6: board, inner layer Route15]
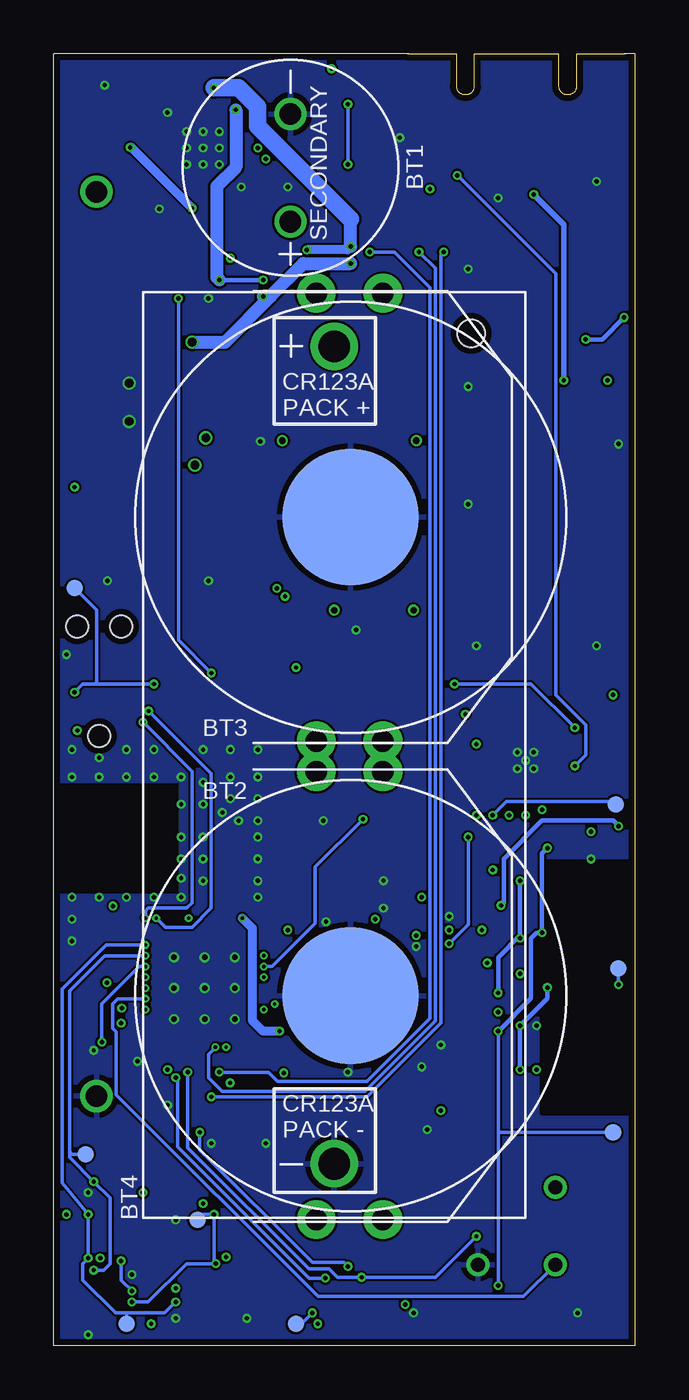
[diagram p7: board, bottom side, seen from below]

Size 27 x 60 mm. Coordinates in mm from the lower left corner, seen from the top.
Outline: 0.5,60 0,60 0,0 27,0 27,60 10.5,60
Copper layers (1+2*15+16): Top 0.0178mm / dielectric 59mil / Route2 0.0356mm / dielectric 0.1499mm / Route15 0.0356mm / dielectric 0.2007mm / Bottom 0.0178mm
Design rules "quickturn_co_kr_1oz_4lyr *": minimum track width 4mil, minimum drill 8mil, track to track 4mil, track to pad 4mil, pad to pad 4mil, via to via 4mil, smd to smd 4mil, copper to edge 12mil, drill to drill 12mil, minimum pad ring 8mil, minimum via ring 4mil, stop-mask expansion 3mil, vias tented up to drill 50mil, thermal gap 10mil
tKeepout: area 13.4,0.8 to 13.5,1.3
tRestrict: area 11.9,1.8 to 12.4,1.8; area 11.9,1.3 to 12.4,1.3; area 12.4,0.8 to 12.5,1.3; area 20.1,1 to 20.2,1.5

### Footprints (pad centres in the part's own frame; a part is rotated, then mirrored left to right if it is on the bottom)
ANT3216A063R2400A = smd 0.6 x 1.8: S1 -1.325,0; S2 1.325,0
1020 = drill 1: + -2.5,0; - 2.5,0
BAT-HLD-002-THM = smd 6.35 x 6.35: GND 0,0 | drill 1 pad 1.8: POS1 -10.4,1.5; POS2 -10.4,-1.6; POS3 10.4,1.5; POS4 10.4,-1.6
BH123A = drill 1.47: + 18.985,0; - -18.985,0 | hole 1.27: 19.58,-6.37
0402_CAP = smd 0.536 x 0.546: 1 -0.433,0; 2 0.433,0
0603_CAP = smd 0.7 x 1: 1 -0.65,0; 2 0.65,0
SOLAR_HOLES = drill 1: + 0,0; - 42,0
1MM_SQ_4PAD = smd 0.457 x 0.457: 1 0.432,0.432; 2 0.432,-0.432; 3 -0.432,-0.432; 4 -0.432,0.432
TC2030-IDC-NL = smd 0.787 x 0.787: 1 -1.27,-0.635; 2 -1.27,0.635; 3 0,-0.635; 4 0,0.635; 5 1.27,-0.635; 6 1.27,0.635 | hole 1.016: -2.54,0; 2.54,1.016; 2.54,-1.016
MICRO_USB_B_HIROSE_ZX62R-B-5P(30) = smd 0.4 x 1.35: 1 1.3,4.125; 2 0.65,4.125; 3 0,4.125; 4 -0.65,4.125; 5 -1.3,4.125 | smd 2.1 x 2: P$1 3.1,3.8; P$2 -3.1,3.8 | smd 1.6 x 1.9: P$3 -4.1,1.45; P$6 4.1,1.45 | smd 1.2 x 1.9: P$4 -0.85,1.45; P$5 0.85,1.45
IHL-1212BZ-11 = smd 1.2 x 1.5: P$1 -1.35,0; P$2 1.35,0
74437324220 = smd 1.5 x 2.4: P$1 1.85,0; P$2 -1.85,0
XDFN-6 = smd 0.35 x 0.2: 1 -0.425,0.35; 2 -0.425,0; 3 -0.425,-0.35; 4 0.425,-0.35; 5 0.425,0; 6 0.425,0.35
0402_RES = smd 0.536 x 0.546: 1 -0.433,0; 2 0.433,0
0603-RES = smd 0.7 x 1: 1 -0.65,0; 2 0.65,0
EVQP2 = smd 1.676 x 0.813: P$1 -2.54,-0.87; P$2 -2.54,0.908; P$3 2.54,-0.87; P$4 2.54,0.908
SJ_2S-NOTRACE = smd 0.635 x 1.27: 1 -0.401,0; 2 0.413,0
PAD.03X.03 = smd 0.762 x 0.762: P$1 0,0
QFN-16-3MM = smd 0.7 x 0.25: 1 -1.4,0.75; 2 -1.4,0.25; 3 -1.4,-0.25; 4 -1.4,-0.75; 9 1.35,-0.75; 10 1.35,-0.25; 11 1.35,0.25; 12 1.35,0.75 | smd 0.25 x 0.7: 5 -0.75,-1.4; 6 -0.25,-1.4; 7 0.25,-1.4; 8 0.75,-1.4; 13 0.75,1.4; 14 0.25,1.4; 15 -0.25,1.4; 16 -0.75,1.4 | smd 1.45 x 1.45: GND 0,0
S-PVQFN-N20-RGR = smd 0.28 x 0.85: 1 -1,-1.74; 2 -0.5,-1.74; 3 0,-1.74; 4 0.5,-1.74; 5 1,-1.74; 11 1,1.74; 12 0.5,1.74; 13 0,1.74; 14 -0.5,1.74; 15 -1,1.74 | smd 0.85 x 0.28: 6 1.74,-1; 7 1.74,-0.5; 8 1.74,0; 9 1.74,0.5; 10 1.74,1; 16 -1.74,1; 17 -1.74,0.5; 18 -1.74,0; 19 -1.74,-0.5; 20 -1.74,-1 | smd 2.05 x 2.05: PAD 0,0
AMN2 = drill 0.65: GND 1.796,-1.796; OUT -1.796,-1.796; VCC -1.796,1.796
QFN32 = smd 0.6 x 0.3: 1 -2.3,1.75; 2 -2.3,1.25; 3 -2.3,0.75; 4 -2.3,0.25; 5 -2.3,-0.25; 6 -2.3,-0.75; 7 -2.3,-1.25; 8 -2.3,-1.75; 17 2.3,-1.75; 18 2.3,-1.25; 19 2.3,-0.75; 20 2.3,-0.25; 21 2.3,0.25; 22 2.3,0.75; 23 2.3,1.25; 24 2.3,1.75 | smd 0.3 x 0.6: 9 -1.75,-2.3; 10 -1.25,-2.3; 11 -0.75,-2.3; 12 -0.25,-2.3; 13 0.25,-2.3; 14 0.75,-2.3; 15 1.25,-2.3; 16 1.75,-2.3; 25 1.75,2.3; 26 1.25,2.3; 27 0.75,2.3; 28 0.25,2.3; 29 -0.25,2.3; 30 -0.75,2.3; 31 -1.25,2.3; 32 -1.75,2.3 | smd 3.2 x 3.2: EXP 0,0
LGA-12 = smd 0.375 x 0.35: 1 -0.75,0.75; 2 -0.75,0.25; 3 -0.75,-0.25; 4 -0.75,-0.75; 7 0.75,-0.75; 8 0.75,-0.25; 9 0.75,0.25; 10 0.75,0.75 | smd 0.35 x 0.375: 5 -0.25,-0.75; 6 0.25,-0.75; 11 0.25,0.75; 12 -0.25,0.75
UDFN-6-MAXIM = smd 0.8 x 0.35: 1 -0.915,0.65; 2 -0.915,0; 3 -0.915,-0.65; 4 0.915,-0.65; 5 0.915,0; 6 0.915,0.65
UDFN-6-EXPOSED = smd 0.48 x 0.36: 1 -0.925,0.65; 2 -0.925,0; 3 -0.925,-0.65; 4 0.925,-0.65; 5 0.925,0; 6 0.925,0.65 | smd 0.71 x 1.4: EP 0,0
4-SMD = smd 1 x 1: 1 -1,1; 2 -1,-1; 3 1,-1; 4 1,1
AQFN73 = smd 0.3 x 0.3: A8 -1.25,3.25; A10 -0.75,3.25; A12 -0.25,3.25; A14 0.25,3.25; A16 0.75,3.25; A18 1.25,3.25; A20 1.75,3.25; A22 2.25,3.25; A23 2.75,3.25; AA24 3.25,-2.25; AB2 -2.75,-2.5; AC5 -2,-2.75; AC9 -1,-2.75; AC11 -0.5,-2.75; AC13 0,-2.75; AC15 0.5,-2.75; AC17 1,-2.75; AC19 1.5,-2.75; AC21 2,-2.75; AC24 3.25,-2.75; AD2 -2.75,-3.25; AD4 -2.25,-3.25; AD6 -1.75,-3.25; AD8 -1.25,-3.25; AD10 -0.75,-3.25; AD12 -0.25,-3.25; AD14 0.25,-3.25; AD16 0.75,-3.25; AD18 1.25,-3.25; AD20 1.75,-3.25; AD22 2.25,-3.25; AD23 2.75,-3.25; B1 -3.25,2.75; B3 -2.5,2.75; B5 -2,2.75; B7 -1.5,2.75; B9 -1,2.75; B11 -0.5,2.75; B13 0,2.75; B15 0.5,2.75; B17 1,2.75; B19 1.5,2.75; B24 3.25,2.75; C1 -3.25,2.25; D2 -2.75,2; D23 2.75,2; E24 3.25,1.75; F2 -2.75,1.5; F23 2.75,1.5; G1 -3.25,1.25; H2 -2.75,1; H23 2.75,1; J1 -3.25,0.75; J24 3.25,0.75; K2 -2.75,0.5; L1 -3.25,0.25; L24 3.25,0.25; M2 -2.75,0; N1 -3.25,-0.25; N24 3.25,-0.25; P2 -2.75,-0.5; P23 2.75,-0.5; R1 -3.25,-0.75; R24 3.25,-0.75; T2 -2.75,-1; T23 2.75,-1; U1 -3.25,-1.25; U24 3.25,-1.25; V23 2.75,-1.5; W1 -3.25,-1.75; W24 3.25,-1.75; Y2 -2.75,-2; Y23 2.75,-2 | smd 4.85 x 4.85: GND 0,0
DFN-6/3MM = smd 0.85 x 0.45: 1 -1.45,1; 2 -1.45,0; 3 -1.45,-1; 4 1.45,-1; 5 1.45,0; 6 1.45,1 | smd 1.6 x 2.5: P$1 0,0
FN-6 = smd 1 x 0.4: 1 -0.75,0.65; 2 -0.75,0; 3 -0.75,-0.65; 4 0.75,-0.65; 5 0.75,0; 6 0.75,0.65
TXC-7V = smd 1.4 x 1.2: 1 -1.1,-0.85; 2 1.1,-0.85; 3 1.1,0.85; 4 -1.1,0.85
ABS05 = smd 0.5 x 1: A -0.55,0; B 0.55,0
2-SMD = smd 1.092 x 1.905: 1 -1.245,0; 2 1.245,0

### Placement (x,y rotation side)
A2  25.31,23.19 270 top
BT1  16,54.7 90 bottom
BT2  13.21,16.26 270 bottom
BT3  13.21,38.48 270 bottom
BT4  13.97,27.43 90 bottom
C1  18.73,23.33 180 top
C2  18.73,20.79 180 top
C3  11.68,22.86 90 top
C4  13.21,19.68 0 top
C5  19.05,10.67 90 top
C6  18.03,9.4 90 top
C7  7.87,29.97 0 top
C8  16.75,21.89 90 top
C9  24.64,57.75 0 top
C10  19.3,51.82 270 top
C11  14.06,14.95 90 top
C12  24.73,19.77 0 top
C13  25.15,16 270 top
C14  16.73,11.52 270 top
C15  15.21,19.27 90 top
C16  23.24,4.7 90 top
C17  16.76,2.29 0 top
C18  7.37,20.32 0 top
C19  7.37,21.34 0 top
C20  7,52.71 90 top
C21  15.72,11.52 270 top
C22  15.34,14.95 90 top
C23  22.23,4.7 90 top
C24  21.21,4.7 90 top
C25  7.62,28.7 0 top
C26  21.21,11.81 180 top
C27  18.29,51.82 270 top
C28  25.15,56.15 0 top
C29  18.8,46.99 180 top
C30  18.8,41.02 180 top
C31  16.51,1.02 0 top
C32  1.78,31.24 90 top
C33  7.37,31.24 90 top
D1  25.02,53.59 270 top
D2  15.11,58.93 90 top
J1  24.89,30.86 90 top
J5  5.5,60 180 top
L1  19.24,22.06 270 top
L2  13.3,13.93 270 top
L3  25.02,43.69 270 top
L4  14.83,13.42 0 top
L5  22.86,50.26 180 top
Q1  5.33,13.84 90 top
Q2  5.33,19.94 270 top
Q3  19.56,5.08 270 top
Q4  25.4,5.08 90 top
Q5  14.22,51.02 0 top
Q6  18.29,49.5 0 top
Q7  22.35,2.03 0 top
Q8  5.33,16.38 0 top
Q10  8,11.81 180 top
R1  12.32,51.94 270 top
R2  8.89,51.94 270 top
R3  10.54,51.94 270 top
R4  19.56,59.18 0 top
R6  1.21,23.23 0 top
R7  2.98,23.23 180 top
R8  23.88,7.75 180 top
R9  21.34,6.6 0 top
R10  8.89,53.98 270 top
R11  2.03,28.96 90 top
R12  0.89,28.96 90 top
R13  18.8,43.81 0 top
R14  22.1,59.18 180 top
R17  17.53,56.77 90 top
R18  16.13,54.99 90 top
R21  22.61,57.91 90 top
R22  18.8,45.21 180 top
R23  23.88,6.6 180 top
R24  17.78,3.81 270 top
R25  7.11,18.54 180 top
R26  5.59,22.61 0 top
R27  9.65,11.3 270 top
S1  12.45,56.26 270 top
SJ2  1.27,45.97 90 top
SJ3  1.27,43.69 90 top
SJ4  5.33,45.97 270 top
SJ5  3.3,45.97 270 top
TP1  1.02,9.91 0 bottom
TP2  1.02,25.15 0 top
TP3  10.67,0.76 180 top
TP4  1.02,9.91 0 top
TP5  11.94,3.43 0 top
TP6  7.87,27.18 0 top
TP7  13.97,4.45 0 top
TP8  7.87,17.27 0 top
TP9  23.62,1.02 0 bottom
TP10  20.32,5.84 0 bottom
TP11  18.16,7.62 0 top
TP12  0.76,17.53 0 bottom
TP13  10.16,23.88 0 top
TP14  3.05,25.91 0 top
TP15  0.89,25.15 0 bottom
TP16  2.03,25.15 0 top
TP17  26.04,35.18 0 bottom
TP18  25.45,13 0 top
TP19  15.75,1.02 0 bottom
TP20  25.53,8.89 0 bottom
TP21  22.61,7.87 0 top
TP22  9.4,0.76 0 top
TP23  23.37,53.85 0 top
TP24  13.84,16.76 0 top
TP25  23.24,41.15 0 top
TP26  26.04,39.12 0 top
TP27  26.04,37.08 0 top
U1  5.08,27.18 0 top
U2  20.07,55.59 90 top
U3  5.5,5.56 0 top
U4  3.43,50.47 90 top
U6  12.95,1.78 270 top
U7  21.84,43.81 90 top
U8  19.81,2.16 90 top
U9  2.03,13.34 90 top
U10  19.99,16.61 90 top
U11  2.02,19.88 270 top
U12  25.15,2.16 0 top
U$2  [UCB_CAL_200MIL]  0.64,37.85 0 top
X1  13.68,22.19 90 top
X3  18.03,11.18 90 top
X4  4.57,30.73 0 top

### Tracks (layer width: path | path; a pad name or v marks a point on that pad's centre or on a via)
!CLR_EN  (via drill 0.15, 0.2)
  Top 0.152: Q7.2 v21.34,2.03 | v25.4,4.06 Q4.2 | Q4.5 v25.4,6.1
  Top 0.254: R23.1 24.89,6.6 v25.4,6.1
  Bottom 0.152: v21.34,2.03 21.84,1.52 23.62,1.52 | 23.62,1.52 24.13,1.52 25.65,3.05 25.65,3.81 v25.4,4.06 v25.4,6.1 26.62,7.57 26.62,16.56 24.57,18.61 U10.AC21 | TP9.P$1 23.62,1.52
  other vias: 22.74,18.61
!CLR_INT  (via drill 0.15, 0.2)
  Top 0.152: U12.5 25.4,2.16 25.15,2.41 v25.15,3.5
  Top 0.203: v25.15,7.62 25.02,7.75 R8.1
  Bottom 0.152: v25.15,3.5 24.69,3.5 24.38,3.81 24.38,6.86 v25.15,7.62 26.26,8.74 26.26,9.02 | U10.AC19 24.64,18.11 26.26,16.48 26.26,9.02 | TP20.P$1 26.14,8.89 26.26,9.02
  other vias: 22.74,18.11
!FTDI_RESET  (via drill 0.2)
  Top 0.203: U4.18 4.68,53.45 v4.7,53.47
  Top 0.254: SJ3.2 2.57,44.1 v3.3,44.83
  Bottom 0.254: v3.3,44.83 3.3,52.07 v4.7,53.47
!HUM_EN  (via drill 0.2)
  Top 0.152: U10.A20 13.26,18.36 12.06,19.56 v12.06,19.81
  Top 0.203: Q2.5 v5.33,18.92 | Q8.5 v6.35,16.38 | Q2.2 v5.33,21.59 5.33,22.43 R26.1
  Route2 0.152: v12.06,19.81 10.29,19.81 8.51,21.59 v5.33,21.59 | v5.33,18.92 3.17,16.76 v0.76,16.76
  Bottom 0.152: v0.76,16.76 TP12.P$1
  Bottom 0.203: v5.33,21.59 5.33,19.05 | 5.33,19.05 v5.33,18.92 | 5.33,19.05 6.35,18.03 v6.35,16.38
!LT_EN  (via drill 0.2)
  Top 0.152: Q3.5 19.56,3.89 v19.48,3.81 | Q7.5 v23.37,2.03 | Q3.2 v19.56,6.1 | R24.1 17.78,4.83 19.05,6.1 v19.56,6.1 | U10.AD20 25.27,18.36 26.29,17.34 26.29,11.05 23.88,8.64 21.49,8.64 19.63,6.78 19.63,6.17 v19.56,6.1
  Bottom 0.152: v19.48,3.81 19.56,3.81 | 19.56,3.81 v19.56,6.1 20.07,6.1 TP10.P$1 | v23.37,2.03 22.61,2.03 20.83,3.81 19.56,3.81
!LT_INT
  Top 0.152: U10.AD22 25.29,18.86 26.54,17.6 26.54,10.92 24,8.38 22.68,8.38 22.17,7.87 | 22.17,7.87 R9.1 20.57,6.28 20.57,3.2 U8.4 | 22.17,7.87 TP21.P$1 22.61,8.13
  Top 0.203: R9.1 20.83,6.68
!PIR_EN
  Top 0.152: U10.AD12 23.77,16.36 24.26,15.88 24.26,13.13 19.51,8.38 18.16,8.38 | R27.1 14.04,11.74 17.4,8.38 18.16,8.38 | TP11.P$1 18.16,8.38
  Top 0.203: Q10.2 9.58,11.81 R27.1
!PR_EN  (via drill 0.15 pad 0.3, 0.2)
  Top 0.152: v6.86,17.78 7.37,17.27 TP8.P$1 | R25.1 8.43,19.3 v8.64,19.3
  Top 0.203: Q1.5 v5.33,14.86 | Q1.2 v5.33,12.83 | Q8.2 4.32,16.38 v4.06,16.64 3.81,16.89 3.81,17.53 4.06,17.78 v6.86,17.78 7.54,18.47 R25.1
  Route2 0.152: U10.B19 9.96,18.11 v8.64,19.3
  Bottom 0.203: v5.33,12.83 v5.33,14.86 4.06,16.13 v4.06,16.64
  other vias: 17.24,18.11
!RST  (via drill 0.15, 0.2)
  Top 0.152: U1.1 2.63,27.93 R11.1 2.62,28.52 v2.79,28.7 | v22.35,30.73 v8.38,30.73 8.38,36.17 SJ3.1
  Top 0.305: J1.3 v26.04,30.35
  Route15 0.152: 22.81,16.61 U10.AC13 22.91,16.61 23.2,16.9 23.2,20 22.88,20.32 20.83,20.32 20.57,20.57 20.57,28.96 v22.35,30.73
  Bottom 0.152: v2.79,28.7 4.83,30.73 v8.38,30.73 | TP17.P$1 25.02,34.16 25.02,30.73 | v22.35,30.73 25.02,30.73 | 25.02,30.73 25.65,30.73 v26.04,30.35
  other vias: 22.74,16.61
!RTC_EXTR  (via drill 0.2)
  Top 0.152: U1.3 v2.8,26.93 v2.79,26.92 | S1.P$2 13.34,58.78 v13.34,57.66 13.08,57.66 9.83,54.41 R10.1 8.84,54.36 v8.26,54.36 | v13.34,54.86 13.34,53.74 S1.P$4
  Bottom 0.152: v2.79,26.92 2.29,27.43 2.29,28.83 3.68,30.23 3.68,49.78 v8.26,54.36 | v13.34,54.86 v13.34,57.66
!RTC_IRQ1
  Top 0.152: U1.11 6.58,27.28 6.88,27.28 7.11,27.04 7.11,25.91 9.65,23.37 | 9.65,23.37 11.18,21.84 11.18,20.07 13.21,18.03 16.04,18.03 16.71,17.36 U10.A16 | TP13.P$1 9.65,23.37
!RTC_IRQ2  (via drill 0.15, 0.2)
  Top 0.152: U1.4 3.68,25.91 | 3.68,25.91 3.68,24.82 4.67,23.82 7.54,23.82 v7.75,23.62 | TP14.P$1 3.68,25.91
  Route2 0.152: U10.B15 10.2,17.11 v8.64,18.67
  Bottom 0.152: v7.75,23.62 7.75,19.56 v8.64,18.67
  other vias: 17.24,17.11
!RTC_IRQ3  (via drill 0.2)
  Top 0.152: U1.8 5.83,25.41 v6.6,24.64 7.11,24.13 8.38,24.13 10.67,21.84 10.67,20.19 13.13,17.73 15.84,17.73 16.71,16.86 U10.A14
  Bottom 0.152: v6.6,24.64 5.97,25.27 1.02,25.27 TP15.P$1
!VBAT_PRI_ON  (via drill 0.2)
  Top 0.203: Q6.2 v17.27,49.5 | Q6.5 v19.3,49.5 | U2.10 19,57.4
  Top 0.406: 19,57.4 v18.54,57.4
  Bottom 0.203: v17.27,49.5 v19.3,49.5
  Bottom 0.61: v19.3,49.5 19.43,49.62 19.43,53.85 18.54,54.74 v18.54,57.4
!VBAT_SEC_ON  (via drill 0.2)
  Top 0.152: Q5.2 13.24,51.02 v13.21,51.05 | Q5.5 15.11,51.02 v15.24,50.9
  Top 0.406: U2.9 v19.57,58.41 v19.56,58.42
  Bottom 0.406: v13.21,51.05 13.37,50.9 v15.24,50.9
  Bottom 0.61: v13.21,51.05 13.21,52.32
  Bottom 0.813: v19.56,58.42 18.41,58.42 17.53,57.54 17.53,56.64 13.21,52.32
ACC_CS  (via drill 0.15, 0.2)
  Top 0.152: U6.2 13.3,2.62 13.3,2.81 14.43,3.94 | 14.43,3.94 15.49,3.94 24.77,13.21 v24.77,14.1 | TP7.P$1 13.97,4.39 14.43,3.94
  Bottom 0.152: 22.78,17.61 U10.AC17 23.03,17.61 24.77,15.88 v24.77,14.1
  other vias: 22.74,17.61
ACC_INT1
  Top 0.152: U6.12 14.02,2.03 21.29,9.3 22.35,9.3 24,10.95 24,11.94 25.07,13 TP18.P$1 25.65,13 25.65,17.09 25.39,17.36 U10.AD16
ACC_INT2  (via drill 0.2)
  Top 0.152: U6.11 13.8,1.62 14.04,1.62 | 14.04,1.62 21.41,8.99 23.85,8.99 26.04,11.18 26.04,17.14 25.32,17.86 U10.AD18 | 14.04,1.62 14.89,1.62 v14.99,1.52
  Bottom 0.152: v14.99,1.52 15.49,1.02 TP19.P$1
D+
  Top 0.203: J5.3 5.5,54.67 5.84,54.32 7.62,54.32 8,53.94 8,51.82 7.4,51.22 U4.14
D-
  Top 0.203: J5.2 4.85,54.3 5.33,53.82 7.37,53.82 7.62,53.56 7.62,51.94 7.39,51.72 U4.15
DBG_RX  (via drill 0.2)
  Top 0.152: U10.G1 18.74,12.27 v18.81,12.2 | SJ5.2 15.75,33.12 v15.75,31.5
  Route2 0.152: v18.81,12.2 18.81,13.45 17.78,14.48 17.78,18.29 15.75,20.32 v15.75,31.5
DBG_TX  (via drill 0.15, 0.2)
  Top 0.152: SJ4.2 16.1,34.8 v16.26,34.8
  Top 0.203: SJ4.2 5.49,45.56
  Route2 0.152: U10.H2 18.09,14.77 18.09,18.41 16.26,20.24 v16.26,34.8
  other vias: 18.99,13.86
FTDI_VCCIO
  Top 0.254: U4.1 1.68,46.8 SJ2.2
GND  (via drill 0.2, 0.25, 0.41)
  Top 0.102: 18.53,18.64 18.53,18.63 | U10.F23 18.49,19.57 18.62,19.7 18.62,20.47 C2.2
  Top 0.203: C1.2 17.84,23.33 | U10.B7 17.9,15.11 | 17.9,15.11 18.03,15.24 | U10.GND 18.49,15.11 17.9,15.11 | U10.F23 18.49,18.54 | 18.49,18.54 18.49,18.14 v18.59,18.03 | U10.GND 19.99,17.04 18.49,18.54 | U10.GND 19.99,17.18 18.53,18.64 | 5.59,47.5 5.08,47.5 4.97,47.6 3.54,47.6 3.18,47.96 U4.4
  Top 0.254: U6.8 12.7,0.51 12.19,0.51 12.2,0.52 U6.7 12.19,1.02 11.68,1.02 11.68,1.52 | 11.68,1.52 11.69,1.53 U6.6 | 11.68,1.52 11.68,2.03 U6.5 | v17.53,23.62 17.82,23.33 C1.2 | U8.2 19.81,0.69 21.08,0.69
  Top 0.406: U9.4 1.03,15.13 1.27,15.37 4.57,15.37 | C4.1 12.78,21.03 X1.4
  other vias: 18.29,53.82 6.35,53.31 7.75,50.01 10.92,56.1 4.57,14.86 23.5,44.7 23.5,42.93 19.3,56.39 20.07,56.39 20.83,56.39 20.83,55.63 20.07,55.63 19.3,55.63 19.3,54.86 20.07,54.86 20.83,54.86 1.78,54.07 22.1,52.8 19.99,18.03 19.99,16.61 19.99,15.16 18.59,16.61 21.41,16.61 21.41,15.16 21.41,18.03 18.59,15.16 14.48,24.38 5.08,27.18 23.11,13.21 4.7,27.56 5.46,27.56 5.46,26.8 4.7,26.8 19.81,48.64 8.64,19.94 21.34,1.27 21.34,5.84 17.53,20.83 17.53,21.59 17.53,22.61 17.53,24.38 21.08,22.61 21.08,21.72 21.08,20.83 22.35,20.83 23.62,20.83 24.89,20.83 26.16,20.83 21.08,23.62 21.08,25.15 21.08,26.42 18.41,24.38 22.35,26.42 23.62,26.42 24.89,26.42 26.16,26.42 25.15,13.72 19.18,24.77 20.07,25.15 2.03,22.61 18.03,1.27 25.4,7.11 23.37,3.3 25.4,0.51 20.07,23.62 20.07,22.61 20.07,21.59 20.07,26.16 18.8,26.42 17.53,26.42 17.53,25.4 18.8,25.4 26.16,19.81 26.16,18.8 17.53,27.69 18.8,27.69 20.07,27.69 22.35,27.69 23.62,27.69 24.89,27.3 26.16,27.69 10.29,1.52 2.67,1.52 21.72,11.18 17.14,9.4 19.68,9.4 21.72,57.28 24.64,58.55 11.68,21.59 11.68,20.32 14.35,19.68 7.37,32.51 1.78,32.51 13.34,12.7 9.91,12.95 10.16,18.54 9.02,13.97 9.65,10.03 16.13,53.82 7.75,44.55 0.76,41.88 12.95,33.24 7.75,39.08 17.4,42.01 19.81,35.53 24.51,35.53 26.42,32.1
  pour Top (rank 2): 0,60 27,60 27,0 0,0
  pour Bottom (rank 2): 0,60 27,60 27,0 0,0
  pour Top (rank 2, no thermals): 24.55,22.05 26.07,22.05 26.07,20.76 24.55,20.76
  pour Route2 (rank 2): 0,60 0,0 27,0 27,60
LBST  (via drill 0.15, 0.2)
  Top 0.152: L5.P$1 20.9,50.15 21.21,49.84 v21.21,48.64 | U10.AC15
  Top 0.254: U2.20 21.07,52.05 21.08,52.55
  Top 0.406: 21.08,52.55 21.08,50.33 L5.P$1
  Route15 0.152: U10.AC15 21.5,17.11 19.68,18.92 v19.68,31.24
  Bottom 0.152: v21.21,48.64 21.21,32.77 v19.68,31.24
  other vias: 22.74,17.11
LED_BLUE  (via drill 0.15, 0.2)
  Top 0.152: R3.2 10.54,51.31 v10.03,50.8
  Bottom 0.152: U10.K2 19.81,13.54 19.81,12.45 19.18,11.81 12.55,11.81 9.27,15.09 9.27,50.04 v10.03,50.8
  other vias: 19.49,13.86
LED_GREEN  (via drill 0.2)
  Top 0.152: U10.L1 19.74,11.61 v19.68,11.56 | R2.2 v8.89,50.8
  Bottom 0.152: v19.68,11.56 12.45,11.56 9.02,14.99 9.02,50.67 v8.89,50.8
LED_RED  (via drill 0.2)
  Top 0.152: U10.J1 19.24,12.76 v19.3,12.7 | R1.2 v12.32,50.8
  Bottom 0.152: v19.3,12.7 17.02,12.7 16.6,12.28 12.44,12.28 9.53,15.2 9.53,49.15 11.18,50.8 v12.32,50.8
MISO  (via drill 0.2)
  Top 0.152: U6.3 v12.7,3.17 | v20.78,12.7 20.78,13.32 U10.R1 | U1.6 4.83,24.89 v5.08,24.64 | v7.37,5.08 3.81,5.08 1.02,7.87 TP4.P$1
  Route15 0.152: v5.08,24.64 7.62,22.1 7.62,5.33 v7.37,5.08
  Bottom 0.152: v20.78,12.7 20.78,9.19 15.15,3.57 14.21,3.57 13.81,3.17 v12.7,3.17 9.27,3.17 v7.37,5.08
MOSI  (via drill 0.2)
  Top 0.152: 12.27,2.59 U6.4 12.2,3.31 12.32,3.43 | v20.22,9.91 20.22,13.34 U10.N1 | v13.34,3.68 12.57,3.68 12.32,3.43 | U1.9 6.43,25.57 v7.37,24.64 | TP5.P$1 12.32,3.43
  Route15 0.152: v13.34,3.68 9.02,3.68 8.23,4.47 8.23,23.77 v7.37,24.64
  Bottom 0.152: v13.34,3.68 13.53,3.87 14.99,3.87 20.22,9.11 v20.22,9.91
N$2
  Top 0.152: C14.1 17.74,12.96 U10.C1
N$3  (via drill 0.15, 0.2)
  Top 0.203: U10.E24 18.23,19.87 18.2,19.87
  Top 0.254: L2.1 13.45,14.51 C11.1 C22.1 15.43,14.61 v16.51,14.61 U10.B5
  Bottom 0.406: U10.E24 17.78,19.4 17.78,15.11 17.27,14.61 v16.51,14.61
  other vias: 18.24,19.86
N$4
  Top 0.152: 16.75,21.13 16.75,21.43 C8.1
  Top 0.203: U10.D23 17.65,19.71 17.65,20.03 17,20.68 16.75,20.93 16.75,21.43
N$5
  Top 0.102: U10.H23 18.99,19.61 18.89,19.71 18.89,20.52 C2.1
  Top 0.305: 19.24,20.87 C2.1 19.16,21.55 arc-90 L1.2
N$6
  Top 0.305: 25.33,24.5 A2.S1 20.35,24.52 arc90 C1.1 19.16,22.57 arc90 L1.1
N$7
  cutout Route2: 21.24,21.02 26.96,21.02 26.96,26.1 21.24,26.1
N$8
  Top 0.203: C3.2 X1.3 12.83,24.01 13.66,24.84 14.67,24.84 15.39,24.12 15.39,21.71 15.88,21.22 U10.B24
N$9
  Top 0.203: U10.A23 15.05,21.06 15.05,21.09 X1.1 14.53,20.58 C4.2
N$10
  cutout Top: 0,22.48 1.78,22.48 1.78,20.95 2.29,20.95 2.29,22.48 4.32,22.48 4.32,10.79 0,10.79
  cutout Route2: 0,22.48 1.78,22.48 2.29,22.48 4.32,22.48 4.32,10.79 0,10.79
  cutout Route15: 0,22.48 1.78,22.48 2.29,22.48 4.32,22.48 4.32,10.79 0,10.79
  cutout Bottom: 0,22.48 1.78,22.48 2.29,22.48 4.32,22.48 4.32,10.79 0,10.79
N$11
  cutout Top: 19.68,19.3 17.91,19.3 17.91,23.88 19.68,23.88
N$12
  Top 0.203: R13.2 22.1,43.81 22.49,44.21 U7.4
N$13
  Top 0.203: U4.16 6.94,52.22 C20.1
N$14
  Top 0.203: U7.6 20.71,45.21 R22.1
N$15
  Top 0.152: R1.1 12.32,54.48 13.97,56.13 16.26,56.13 16.26,56.15 16.93,56.82 16.93,57.98 D2.2
N$17
  Top 0.152: D2.4 14.68,58.17 11.51,54.99 10.99,54.99 10.29,54.29 10.29,53.77 R2.1
N$18
  Top 0.254: 20.57,57.34 U2.7 20.57,57.78 21.08,58.29 22.55,58.29 R21.2 22.53,58.42 R14.1
N$19
  Top 0.152: D2.3 11.79,54.74 11.1,54.74 10.54,54.18 R3.1
N$20
  Top 0.152: U8.1 19.16,0.52 19.3,0.38 21.46,0.38 21.93,0.84 Q7.3
N$21
  Top 0.203: Q8.6 5.92,16.89 6.6,16.89 7.11,16.38
  Top 0.406: 7.11,16.38 7.11,13.08 5.33,11.3 1.27,11.3 1.02,11.56 1.02,12.32 U9.1
N$22
  Top 0.152: 4.06,16.03 Q8.3
  Top 0.254: 3.4,16.03 4.06,16.03
  Top 0.406: 3.4,16.03 2.02,17.41 U11.5
N$23
  Top 0.203: Q10.6 3.7,7.58 U3.VCC
N$25
  Top 0.203: U1.14 5.33,29.21 5.59,29.46 6.93,29.46 C7.1
N$26
  Top 0.203: U1.16 4.33,29.2 3.33,30.2 X4.1 1.85,30.73 C32.1
N$27
  Top 0.203: U1.15 4.83,29.21 5.59,29.97 5.84,29.97 5.82,30 X4.2 7.29,30.73 C33.1
N$31
  Top 0.152: Q7.6 22.78,2.58 23.11,2.92 24.28,2.92 U12.1
N$32
  Top 0.254: 20.07,57.91 U2.8 20.07,59.18 | R4.2 20.07,59.18 | 20.07,59.18 R14.2
N$34
  Top 0.152: Q1.6
  Top 0.203: U9.3 3.1,14.27 Q1.6
N$35
  cutout Route15: 21.24,21.02 26.96,21.02 26.96,26.1 21.24,26.1
N$38
  cutout Top: 21.24,26.1 26.96,26.1 26.96,23.32 26.96,21.02 26.07,21.02 26.07,22.05 24.55,22.05 24.55,21.02 21.24,21.02
N$39
  cutout Bottom: 21.24,21.02 26.96,21.02 26.96,26.1 21.24,26.1
N$41
  Top 0.203: U9.2 5.6,12.34 5.84,12.57 5.84,13.26 Q1.3
  Top 0.254: 3.05,12.32 U9.2
N$44
  Top 0.254: L4.2 16.57,13.42 16.57,13.44 U10.B3
N$45
  Top 0.152: Q5.1 13.61,51.56 13.08,51.56 12.83,51.31 12.83,50.04 13.08,49.78 13.76,49.78 14.02,50.04 14.48,50.04 14.65,50.21 Q5.4
N$48
  Top 0.152: Q2.3
  Top 0.203: U11.1 4.02,21.32 Q2.3
N$49
  Top 0.254: L4.1 13.38,13.42 L2.2
N$50
  Top 0.152: Q2.6
  Top 0.203: U11.6 3.03,18.41 5.59,18.41 5.84,18.67 5.84,19.36 Q2.6
N$51
  Top 0.152: U8.6 19.14,3.21 18.54,3.81 18.54,5.08 18.97,5.5 Q3.3
N$52
  Top 0.152: Q3.6 19.91,3.31 U8.5
N$53
  Top 0.152: Q6.4
  Top 0.203: Q6.1 17.7,50.01 17.02,50.01 16.76,49.75 16.76,48.57 17.06,48.27 18.33,48.27 18.71,48.65 Q6.4
N$54
  Top 0.152: Q4.3 25.9,4.5 U12.6
N$55  (via drill 0.2)
  Top 0.152: v23.37,2.54 23.5,2.54 23.88,2.16 U12.2 | Q4.6 24.68,5.5 24.38,5.21 24.38,4.45 v23.88,3.94
  Bottom 0.152: v23.88,3.94 23.88,3.05 v23.37,2.54
N$57
  Top 0.254: U2.12 17.77,56.09 R17.1 17.04,56.34 R18.2
N$58
  Top 0.254: R4.1 17.96,58.02 17.96,57.15 | 17.96,57.15 17.96,56.95 U2.11 | R17.2 17.91,57.2 17.96,57.15
PIR_OUT  (via drill 0.15)
  Top 0.152: U3.OUT 6.65,0.81 9.35,0.81 TP22.P$1
  Bottom 0.152: U3.OUT 5.18,2.29 14.73,2.29 24.09,11.64 24.09,14.57 24.26,14.73 24.26,15.88 24.02,16.11 U10.AC11
  other vias: 22.74,16.11
RTC_CS  (via drill 0.15, 0.2)
  Top 0.152: U1.12 6.44,27.94 v7.37,27.94 | 7.87,27.43 TP6.P$1 10.6,24.45 v12.64,24.45
  Top 0.203: v7.37,27.94 7.87,27.43
  Bottom 0.152: U10.B17 16.86,17.61 14.86,19.61 14.86,22.23 v12.64,24.45 12.57,24.51
  other vias: 17.24,17.61
RXD
  Top 0.203: SJ4.1 5.33,46.74 4.83,47.24 2.79,47.24 2.18,47.86 U4.2
SCK  (via drill 0.2)
  Top 0.152: U6.1 13.78,2.53 v14.39,3.14 | U1.7 5.33,25.15 v5.84,24.64 | TP3.P$1 v10.67,1.91 | U10.U1 21.24,12.54 v21.34,12.45
  Route15 0.152: v5.84,24.64 7.92,22.55 7.92,4.27 9.65,2.54 10.67,2.54 | 10.67,2.54 13.79,2.54 v14.39,3.14 | v10.67,1.91 10.67,2.54
  Bottom 0.152: v14.39,3.14 15.15,3.14 21.25,9.23 21.25,12.36 v21.34,12.45
SCL  (via drill 0.15, 0.2)
  Top 0.152: Q4.1 24.84,4.45 v24.84,4.06 | Q2.1 6.14,20.36 v6.22,20.45 | TP2.P$1 1.02,24.38 v0.76,24.13
  Top 0.203: Q1.1 4.57,13.01 v4.57,12.83 | v0.76,24.13 0.76,23.24 R6.1 | Q3.1 20.07,5.66 v20.07,6.6
  Route2 0.152: 22.35,6.66 22.3,6.6 | v20.07,6.6 19.56,7.11 10.29,7.11 v4.57,12.83
  Route2 0.203: v4.57,12.83 4.06,13.34 4.06,14.99 4.12,15.04 4.12,15.05 6.22,17.16 v6.22,20.45 | v24.84,4.06 22.3,6.6 v20.07,6.6
  Route15 0.152: U10.AC9 22.36,15.23 | 22.36,15.23 22.35,15.22 | v20.07,6.6 22.36,8.9 22.36,15.23
  Bottom 0.203: v0.76,24.13 1.02,24.38 4.32,24.38 6.1,22.61 6.1,20.57 v6.22,20.45
  other vias: 22.74,15.61
SDA  (via drill 0.2)
  Top 0.152: 3.56,23.09 R7.1 | Q3.4 19,4.44 v19,4.12 | Q4.4 26.34,6.1 v26.42,6.1 | v23.84,15.68 23.66,15.86 U10.AD10
  Top 0.203: Q2.4 4.65,19.18 v4.32,19.18 | Q1.4 6.02,14.61 v6.35,14.61 | R7.1 3.95,23.23 v4.06,23.11
  Route2 0.152: v6.35,2.79 12.34,2.79 12.52,2.62 17.49,2.62 v19,4.12 | v23.84,15.68 26.42,13.11 v26.42,6.1
  Route2 0.203: v19,4.12 19.01,4.12 19.16,4.27 20.38,4.27 21.79,2.86 21.79,2.85 23.11,1.52 25.65,1.52 26.42,2.29 v26.42,6.1
  Bottom 0.152: v6.35,14.61 6.35,9.91 | 6.35,9.91 v6.35,2.79 | TP1.P$1 6.35,9.91
  Bottom 0.203: v6.35,14.61 4.83,16.13 4.83,18.92 4.57,19.18 v4.32,19.18 4.32,22.86 v4.06,23.11
SW  (via drill 0.2)
  Top 0.152: U10.AD8 23.5,15.36 v23.88,14.99 | v16.64,35.18 22.61,41.15 TP25.P$1
  Route2 0.152: v23.88,14.99 22.35,14.99 16.64,20.7 v16.64,35.18
  pour Top (isolate 0.203, no thermals): 21.72,43.31 21.72,40.39 26.54,40.39 26.54,42.04 21.97,42.04 21.97,43.31
SWDCLK  (via drill 0.15, 0.2)
  Top 0.152: v22.59,29.48 23.98,30.86 J1.4
  Bottom 0.152: U10.AA24 21.81,19.43 20.57,19.43 19.68,20.32 19.68,26.57 v22.59,29.48
  other vias: 22.24,19.86
SWDIO  (via drill 0.15, 0.2)
  Top 0.152: v22.86,28.96 23.5,29.59 J1.2
  Bottom 0.152: U10.AC24 22.74,20.18 22.61,20.32 20.83,20.32 20.57,20.57 20.57,26.67 v22.86,28.96
  other vias: 22.74,19.86
TXD  (via drill 0.2)
  Top 0.203: U4.30 0.69,49.72 0.51,49.53 v0.51,47.75 | v2.29,46.74 2.94,46.74 SJ5.1
  Bottom 0.203: v0.51,47.75 1.52,46.74 v2.29,46.74
USB_5V
  Top 0.203: J5.1 4.31,55.77 4.18,55.64 U4.19
VBAT  (via drill 0.15, 0.2)
  Top 0.152: Q6.6 18.71,50.01 | U1.5 4.33,24.9 v4.32,24.89
  Top 0.203: U10.A10
  Top 0.254: v18.8,50.51 18.71,50.43 18.71,50.01 18.71,49.88 | U2.14 17.17,55.09 v17.14,55.12
  Route15 0.152: U10.A10 16.73,15.88 13.97,15.88
  Route15 0.254: v4.32,24.89 4.57,25.15 10.2,25.15 BT2.POS1
  Route15 0.61: v18.8,50.51 17.27,50.51 | 17.27,50.51 17.24,50.51 15.68,48.96 14.89,48.96 BT3.POS2 | 17.27,50.51 17.27,51.97 17.29,51.98 17.29,54.98 v17.14,55.12
  other vias: 16.74,15.86
  pour Route15: 10.67,49.91 15.88,49.91 15.88,4.7 10.67,4.7
VBAT_OK  (via drill 0.15, 0.2)
  Top 0.152: v17.53,55.63 17.56,55.59 U2.13 | U10.R24
  Route2 0.152: U10.R24 20.57,20.03 20.57,28.96 18.03,31.5 18.03,53.47 17.53,53.98 v17.53,55.63
  other vias: 20.74,19.86
VCC  (via drill 0.2, 0.3, 0.41)
  Top 0.152: Q7.4 22.78,1.31 v22.48,1.02 | Q7.1 21.64,2.67 v21.34,2.67 | TP26.P$1 v26.04,39.88 | v14.1,59.31 14.63,59.31 D2.1 | R10.2 9.35,53.54 v9.53,53.72
  Top 0.203: C12.1 23.56,19.78 23.28,19.5 23.28,19.4 U10.AD23 | 15.22,18.85 C15.1 15.17,18.8 | 16.75,18.85 U10.A22 16.73,18.85 | Q8.1 4.73,16.73 | 7.37,28.7 C25.1 7.11,28.7 5.95,28.7 U1.13 | R11.2 2,29.4 | 2,29.4 1.85,29.46 | C19.1 C18.1 6.68,20.07 6.68,19.3 | R25.2 6.68,19.3 | R6.2 2.03,23.23 | 2.03,23.23 R7.2 | 2.03,23.23 v2.03,23.88 | 6.68,19.3 v7.11,19.3 | U10.Y2 21.96,13.83 | R23.2 R8.2 | 15.85,1.03 C31.1 | U6.9 13.21,0.51 13.72,0.51 13.7,0.52 U6.10 | 25.15,16.26 C13.1 | Q8.4 6.3,15.49 v6.35,15.49 | R12.2 2,29.4 | 9.58,10.87 R27.2 9.6,10.92 v9.02,10.92 8.48,11.46 Q10.1 | U10.W1 21.72,13.34
  Top 0.254: 16.82,12.92 16.82,12.94 U10.B1 | v21.34,2.67 21.21,2.79 C24.1 C23.1 C16.1 23.57,4.27 23.88,4.57 23.88,5.84 23.44,6.28 R23.2 22.86,6.6 | R9.2 22.86,6.6 | U6.10 v14.72,1.03 | v14.72,1.03 14.74,1.03 | 14.74,1.03 15.85,1.03 | C31.1 15.86,1.81 C17.1 16.33,2.62 17.09,3.38 R24.2 | 14.74,1.03 v14.73,1.02 v14.72,1.03 | v22.86,7.11 22.86,6.6 | U10.A22 16.13,18.86 | 16.13,18.86 15.24,18.86 15.22,18.85 | R26.2 6.1,22.61 v6.6,22.1 6.93,21.77 C19.1 | v16.13,19.3 16.13,18.86 | 7.11,28.7 7.12,28.7 7.75,29.33 v7.87,29.33 | R12.2 1.02,29.52 v1.02,30.23 | U10.AD14 v24.54,16.87 24.97,16.43 C13.1 | C12.1 24.3,20.37 v24.25,20.42 | Q8.1 4.91,17.19 4.99,17.27 v5.33,17.27 | v1.27,44.83 SJ2.1
  Top 0.305: 16.82,12.92 16.57,12.92 v16.32,12.66 | v25.91,28.57 25.91,29.21 J1.1
  Top 0.406: C21.1 15.72,12.06 v16.32,12.66 | 21.74,13.61 U10.Y2 21.72,13.59 21.72,13.34 v21.72,12.83 21.72,12.78 21.84,12.66 21.84,12.01 C26.1
  Route2 0.406: v16.13,19.3 15.88,19.05 v10.16,19.05
  Route2 0.813: v16.38,42.04 v10.16,42.04 | v13.97,34.16 v10.29,34.16
  Route15 0.813: v13.97,34.16 15.75,34.16 16.38,33.53
  other vias: 19.94,42.16 20.45,40.89
  pour Top (isolate 0.203, no thermals): 20.32,43.18 21.21,43.18 21.21,40.39 19.3,40.39 19.3,42.67 20.32,42.67
  pour Route15 (rank 2): 0,60 27,60 27,0 0,0
VOC_SAMP_VSTOR  (via drill 0.2)
  Top 0.152: C10.1 19.99,52.25 | Q5.6 15.43,51.37 15.75,51.05 17.09,51.05 C27.1
  Top 0.203: v20.57,52.83 20.57,53.06 U2.19
  Top 0.254: U2.3 21.82,55.61 23.31,55.61 23.35,55.65 v23.45,55.65 | C27.1 19.99,52.25 v20.57,52.83
  Bottom 0.406: v20.57,52.83 23.39,55.65 v23.45,55.65
VREF_SAMP
  Top 0.406: U2.4 22.55,56.09 C9.1
VSEC  (via drill 0.2)
  Top 0.152: U10.A8 16.64,15.36 15.9,16.11 13.84,16.11 | TP24.P$1 13.84,16.11 | 13.84,16.11 13.72,16.11 9.91,19.91 v9.91,20.83
  Top 0.203: U2.18 20.07,53.31 19.81,53.05
  Top 0.406: 19.81,53.05 16.55,53.05 16,52.51 BT1.+
  Route2 0.152: v9.91,20.83 9.53,21.21 9.53,49.4 12.33,52.2 BT1.+
VSOL  (via drill 0.15)
  Top 0.406: U2.2 24.12,55.09 24.13,55.09
  Route15 0.152: U10.B9 17.78,16.15 17.78,19.81 17.02,20.57 17.02,35.56 25.02,43.56 D1.+ 25.02,49.28
  other vias: 17.24,15.61
  pour Top (no thermals): 23.88,56.43 23.88,55.09 22.86,54.07 22.86,48.74 26.16,48.74 26.16,53.82 24.89,55.09 24.89,56.43
VSW  (via drill 0.2, 0.41)
  Top 0.152: v13.21,50.26 13.62,50.67 Q5.3
  Top 0.203: Q6.3 17.45,48.74 v17.27,48.74
  Top 0.305: R22.2 18.15,45.69 C29.1
  Bottom 0.61: 16.92,48.74 v17.27,48.74 | v20.57,46.61 19.05,46.61 16.92,48.74 | 16.92,48.74 15.4,50.26 v13.21,50.26
  pour Top (isolate 0.203, no thermals): 21.72,44.32 21.72,45.85 19.43,45.85 19.43,47.24 26.54,47.24 26.54,45.34 21.97,45.34 21.97,44.32
WDI
  Top 0.152: U1.2 2.29,27.43 | 2.29,27.43 1.98,27.43 R12.1 | 2.29,27.43 2.29,25.7 2.82,25.17 | U10.A12 16.71,16.36 15.67,17.4 12.95,17.4 10.29,20.07 10.29,21.08 8.13,23.24 4.75,23.24 4.47,23.52 2.82,25.17 | TP16.P$1 2.79,25.15 2.82,25.17
XL1
  Top 0.102: U10.D2 17.99,13.61 18.09,13.51 18.09,12.82 17.94,12.67 17.33,12.06 17.33,11.33 X3.A
  Top 0.203: X3.A 17.96,10.55 18.03,10.48 C6.2
XL2
  Top 0.102: U10.F2 18.49,13.61 18.39,13.51 18.39,12.08 X3.B
  Top 0.203: C5.2 18.43,11.73 X3.B

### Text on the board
bPlace: SECONDARY | CR123A / PACK + | CR123A / PACK -
tNames: RESET | SOLAR | VCC | Permamote / Neal Jackson / 6/18 | GND | SOLAR

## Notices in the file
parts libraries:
SparkFun-Passives: Licensing: CC v3.0 Share-Alike You are welcome to use this library for commercial purposes.
